FUNCTION "FC_GRP_71" : VOID
TITLE =GROUP =71
{ S7_language := '9(1) Angielski (Stany Zjednoczone)  11.01.2022  09:45:15' }
VERSION : 0.1


VAR_TEMP
  CL : "UDT_CABINET";	//CABINET LOCAL
  CR : "UDT_CABINET";	//CABINET REMOTE
  RelError : BOOL ;	//ERROR RELEASE
  RelErrorCL : BOOL ;	//ERROR RELEASE FROM CABINET LOCAL
  RelErrorCR : BOOL ;	//ERROR RELEASE FROM CABINET REMOTE
  RelControl : BOOL ;	//CONTROL RELEASE
  RelControlCL : BOOL ;	//CONTROL RELEASE FROM CABINET LOCAL
  RelControlCR : BOOL ;	//CONTROL RELEASE FROM CABINET REMOTE
  ErrorConfirm : BOOL ;	//ERROR CONFIRM
  AutoOn : BOOL ;	//AUTOMATIC ON
  AutoOff : BOOL ;	//AUTOMATIC OFF
  RelAuto : BOOL ;	//AUTOMATIC RELEASE
  TempFlapPos : WORD ;
  TempSetpoint : REAL ;
  LAMP_ON : BOOL ;
  Dummy_bin : BOOL ;
  H_REMAIN : INT ;
  M_REMAIN : INT ;
  S_REMAIN : INT ;
  PosClose : BOOL ;
END_VAR
BEGIN
NETWORK
TITLE =GLOBAL SIGNALS
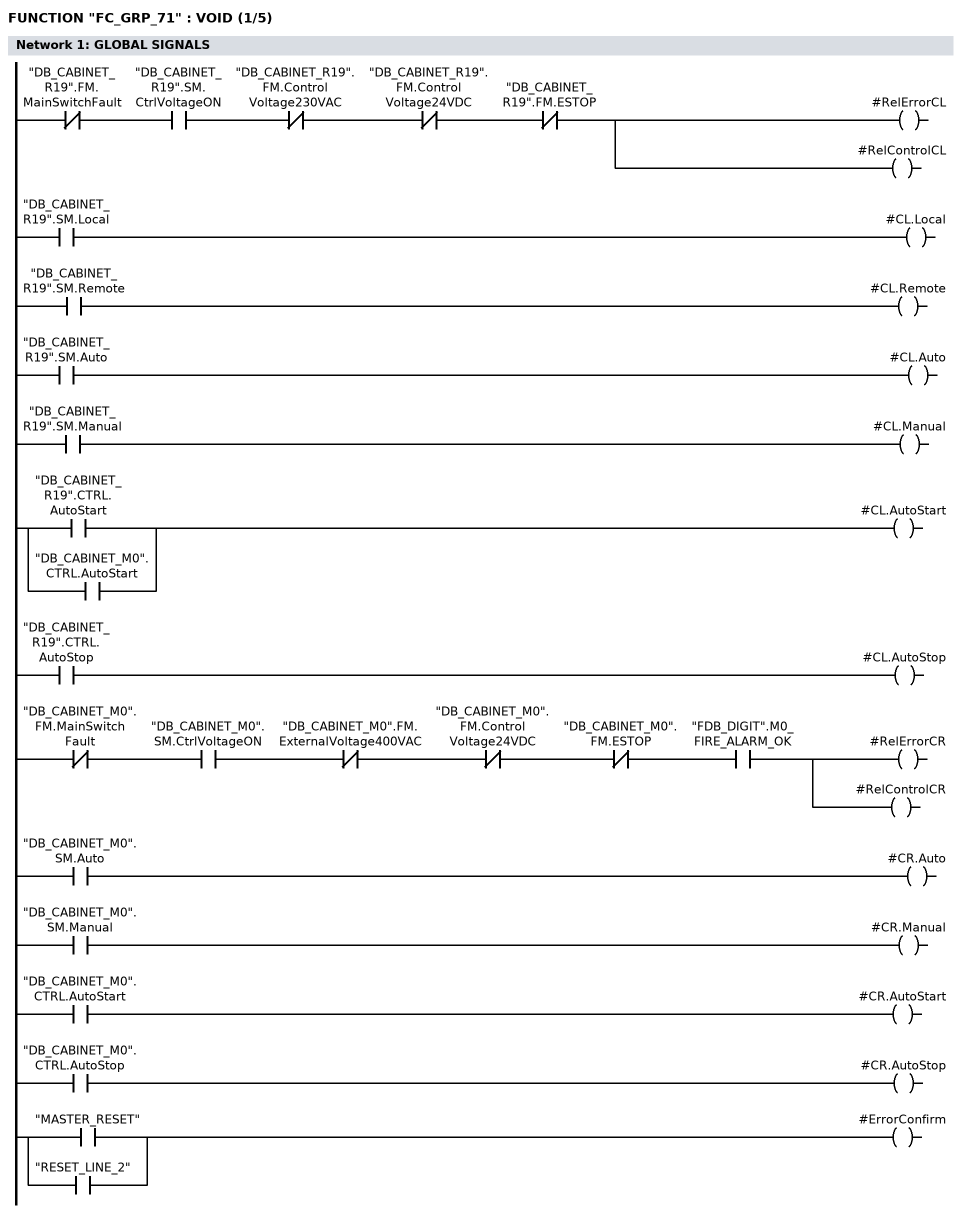
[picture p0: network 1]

//LOCAL
      UN    "DB_CABINET_R19".FM.MainSwitchFault;
      U     "DB_CABINET_R19".SM.CtrlVoltageON;
      UN    "DB_CABINET_R19".FM.ControlVoltage230VAC;
      UN    "DB_CABINET_R19".FM.ControlVoltage24VDC;
      UN    "DB_CABINET_R19".FM.ESTOP;
      =     #RelErrorCL;
      =     #RelControlCL;

      U     "DB_CABINET_R19".SM.Local;
      =     #CL.Local;
      U     "DB_CABINET_R19".SM.Remote;
      =     #CL.Remote;
      U     "DB_CABINET_R19".SM.Auto;
      =     #CL.Auto;
      U     "DB_CABINET_R19".SM.Manual;
      =     #CL.Manual;
      U     "DB_CABINET_R19".CTRL.AutoStart;
      O     "DB_CABINET_M0".CTRL.AutoStart;
      =     #CL.AutoStart;
      U     "DB_CABINET_R19".CTRL.AutoStop;
      =     #CL.AutoStop;


//REMOTE
      UN    "DB_CABINET_M0".FM.MainSwitchFault;
      U     "DB_CABINET_M0".SM.CtrlVoltageON;
      UN    "DB_CABINET_M0".FM.ExternalVoltage400VAC;
      UN    "DB_CABINET_M0".FM.ControlVoltage24VDC;
//      UN    "DB_CABINET_M0".FM.ControlVoltage230VAC_MS
      UN    "DB_CABINET_M0".FM.ESTOP;
      U     "FDB_DIGIT".M0_FIRE_ALARM_OK;
      =     #RelErrorCR;
      =     #RelControlCR;

      U     "DB_CABINET_M0".SM.Auto;
      =     #CR.Auto;
      U     "DB_CABINET_M0".SM.Manual;
      =     #CR.Manual;
      U     "DB_CABINET_M0".CTRL.AutoStart;
      =     #CR.AutoStart;
      U     "DB_CABINET_M0".CTRL.AutoStop;
      =     #CR.AutoStop;

      U     "MASTER_RESET";
      O     "RESET_LINE_2";
      =     #ErrorConfirm;

NETWORK
TITLE =GENERAL ERROR AND WARNING
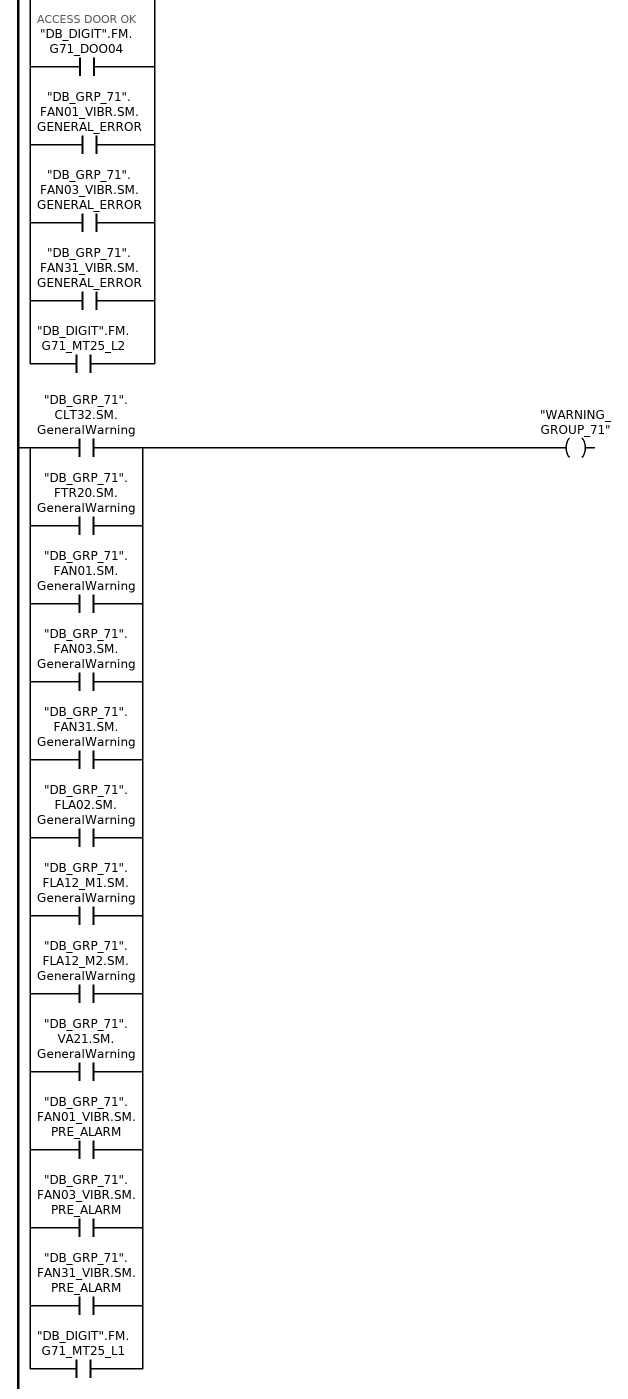
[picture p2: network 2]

      U     "DB_GRP_71".CLT32.SM.GeneralError;
      O     "DB_GRP_71".FTR20.SM.GeneralError;
      O     "DB_GRP_71".FAN01.SM.GeneralError;
      O     "DB_GRP_71".FAN03.SM.GeneralError;
      O     "DB_GRP_71".FAN31.SM.GeneralError;
      O     "DB_GRP_71".FLA02.SM.GeneralError;
      O     "DB_GRP_71".FLA12_M1.SM.GeneralError;
      O     "DB_GRP_71".FLA12_M2.SM.GeneralError;
      O     "DB_GRP_71".VA21.SM.GeneralError;
      O     "DB_DIGIT".FM.G71_FAN01; //ALARM SENSOR PRESSURE
      O     "DB_DIGIT".FM.G71_FAN03; //ALARM SENSOR PRESSURE
      O     "DB_DIGIT".FM.G71_FAN31; //ALARM SENSOR PRESSURE
      O     "DB_DIGIT".FM.G71_DOO01_FUSE; //FUSE ALARM
      O     "DB_DIGIT".FM.G71_DOO02_FUSE; //FUSE ALARM
      O     "DB_DIGIT".FM.G71_DOO03_FUSE; //FUSE ALARM
      O     "DB_DIGIT".FM.G71_DOO04_FUSE; //FUSE ALARM
      O     "DB_DIGIT".FM.G71_DOO04; // ACCESS DOOR OK
      O     "DB_GRP_71".FAN01_VIBR.SM.GENERAL_ERROR;
      O     "DB_GRP_71".FAN03_VIBR.SM.GENERAL_ERROR;
      O     "DB_GRP_71".FAN31_VIBR.SM.GENERAL_ERROR;
      O     "DB_DIGIT".FM.G71_MT25_L2;
      =     "GENERAL_FAULT_GROUP_71";


      U     "DB_GRP_71".CLT32.SM.GeneralWarning;
      O     "DB_GRP_71".FTR20.SM.GeneralWarning;
      O     "DB_GRP_71".FAN01.SM.GeneralWarning;
      O     "DB_GRP_71".FAN03.SM.GeneralWarning;
      O     "DB_GRP_71".FAN31.SM.GeneralWarning;
      O     "DB_GRP_71".FLA02.SM.GeneralWarning;
      O     "DB_GRP_71".FLA12_M1.SM.GeneralWarning;
      O     "DB_GRP_71".FLA12_M2.SM.GeneralWarning;
      O     "DB_GRP_71".VA21.SM.GeneralWarning;
      O     "DB_GRP_71".FAN01_VIBR.SM.PRE_ALARM;
      O     "DB_GRP_71".FAN03_VIBR.SM.PRE_ALARM;
      O     "DB_GRP_71".FAN31_VIBR.SM.PRE_ALARM;
      O     "DB_DIGIT".FM.G71_MT25_L1;
      =     "WARNING_GROUP_71";


NETWORK
TITLE =CONTROL/ERROR RELEASE
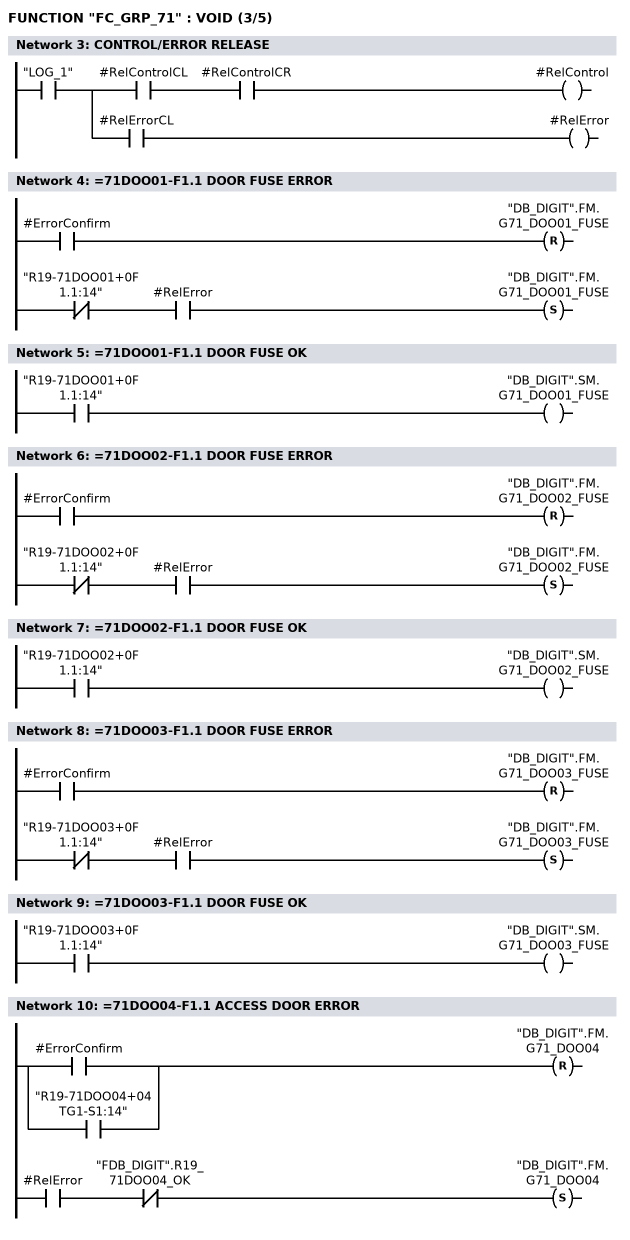
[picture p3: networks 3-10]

      U     "LOG_1";
      =     L     21.0;
      U     L     21.0;
      U     #RelControlCL;
      U     #RelControlCR;
      =     #RelControl;
      U     L     21.0;
      U     #RelErrorCL;
      =     #RelError;
NETWORK
TITLE ==71DOO01-F1.1 DOOR FUSE ERROR

      U     #ErrorConfirm;
      R     "DB_DIGIT".FM.G71_DOO01_FUSE;
      UN    "R19-71DOO01+0F1.1:14";
      U     #RelError;
      S     "DB_DIGIT".FM.G71_DOO01_FUSE;
      NOP   0;
NETWORK
TITLE ==71DOO01-F1.1 DOOR FUSE OK

      U     "R19-71DOO01+0F1.1:14";
      =     "DB_DIGIT".SM.G71_DOO01_FUSE;
NETWORK
TITLE ==71DOO02-F1.1 DOOR FUSE ERROR

      U     #ErrorConfirm;
      R     "DB_DIGIT".FM.G71_DOO02_FUSE;
      UN    "R19-71DOO02+0F1.1:14";
      U     #RelError;
      S     "DB_DIGIT".FM.G71_DOO02_FUSE;
      NOP   0;
NETWORK
TITLE ==71DOO02-F1.1 DOOR FUSE OK

      U     "R19-71DOO02+0F1.1:14";
      =     "DB_DIGIT".SM.G71_DOO02_FUSE;
NETWORK
TITLE ==71DOO03-F1.1 DOOR FUSE ERROR

      U     #ErrorConfirm;
      R     "DB_DIGIT".FM.G71_DOO03_FUSE;
      UN    "R19-71DOO03+0F1.1:14";
      U     #RelError;
      S     "DB_DIGIT".FM.G71_DOO03_FUSE;
      NOP   0;
NETWORK
TITLE ==71DOO03-F1.1 DOOR FUSE OK

      U     "R19-71DOO03+0F1.1:14";
      =     "DB_DIGIT".SM.G71_DOO03_FUSE;
NETWORK
TITLE ==71DOO04-F1.1 ACCESS DOOR ERROR

      U(    ;
      O     #ErrorConfirm;
      O     "R19-71DOO04+04TG1-S1:14";
      )     ;
      R     "DB_DIGIT".FM.G71_DOO04;
      U     #RelError;
      UN    "FDB_DIGIT".R19_71DOO04_OK;
      S     "DB_DIGIT".FM.G71_DOO04;
      NOP   0;
NETWORK
TITLE =DOOR ACKNOWLEDGEMENT
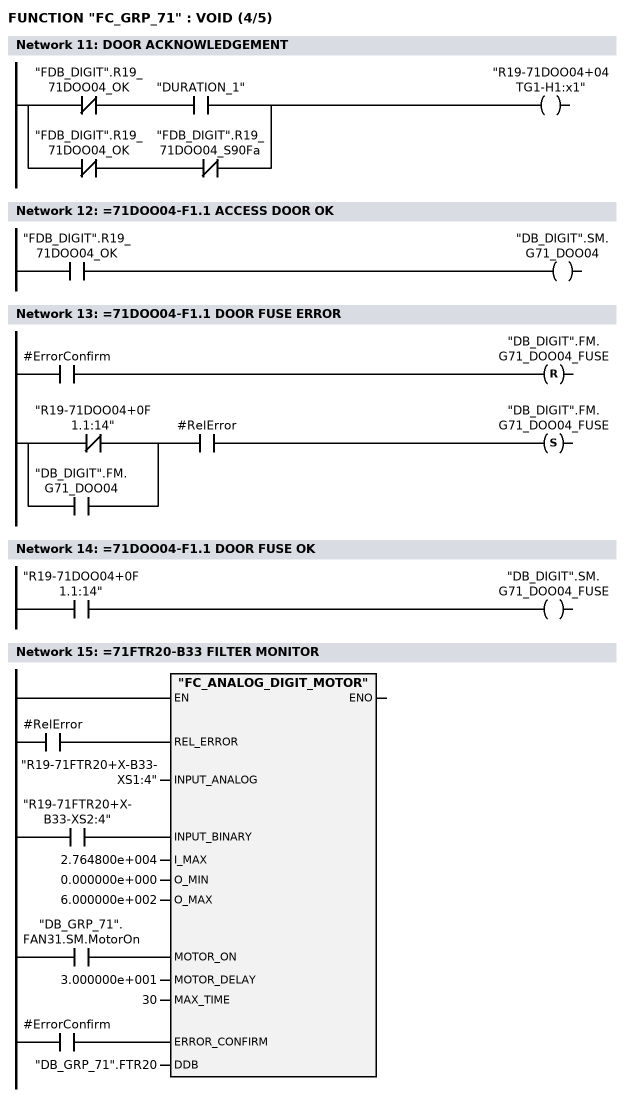
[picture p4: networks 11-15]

      UN    "FDB_DIGIT".R19_71DOO04_OK;
      U     "DURATION_1";
      O     ;
      UN    "FDB_DIGIT".R19_71DOO04_OK;
      UN    "FDB_DIGIT".R19_71DOO04_S90Fa;
      =     "R19-71DOO04+04TG1-H1:x1";
NETWORK
TITLE ==71DOO04-F1.1 ACCESS DOOR OK

      U     "FDB_DIGIT".R19_71DOO04_OK;
      =     "DB_DIGIT".SM.G71_DOO04;
NETWORK
TITLE ==71DOO04-F1.1 DOOR FUSE ERROR

      U     #ErrorConfirm;
      R     "DB_DIGIT".FM.G71_DOO04_FUSE;
      U(    ;
      ON    "R19-71DOO04+0F1.1:14";
      O     "DB_DIGIT".FM.G71_DOO04;
      )     ;
      U     #RelError;
      S     "DB_DIGIT".FM.G71_DOO04_FUSE;
      NOP   0;
NETWORK
TITLE ==71DOO04-F1.1 DOOR FUSE OK

      U     "R19-71DOO04+0F1.1:14";
      =     "DB_DIGIT".SM.G71_DOO04_FUSE;
NETWORK
TITLE ==71FTR20-B33 FILTER MONITOR

      U     #RelError;
      =     L     21.0;
      BLD   103;
      U     "R19-71FTR20+X-B33-XS2:4";
      =     L     21.1;
      BLD   103;
      U     "DB_GRP_71".FAN31.SM.MotorOn;
      =     L     21.2;
      BLD   103;
      U     #ErrorConfirm;
      =     L     21.3;
      BLD   103;
      CALL "FC_ANALOG_DIGIT_MOTOR" (
           REL_ERROR                := L     21.0,
           INPUT_ANALOG             := "R19-71FTR20+X-B33-XS1:4",
           INPUT_BINARY             := L     21.1,
           I_MAX                    := 2.764800e+004,
           O_MIN                    := 0.000000e+000,
           O_MAX                    := 6.000000e+002,
           MOTOR_ON                 := L     21.2,
           MOTOR_DELAY              := 3.000000e+001,
           MAX_TIME                 := 30,
           ERROR_CONFIRM            := L     21.3,
           DDB                      := "DB_GRP_71".FTR20);
      NOP   0;
NETWORK
TITLE ==71CLT32-B40N TEMPERATURE EXCEEDED
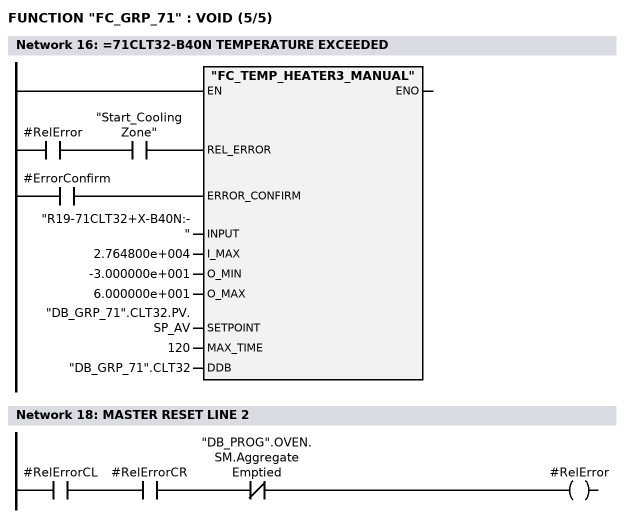
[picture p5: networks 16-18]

      U     #RelError;
      U     "Start_CoolingZone";
      =     L     21.0;
      BLD   103;
      U     #ErrorConfirm;
      =     L     21.1;
      BLD   103;
      CALL "FC_TEMP_HEATER3_MANUAL" (
           REL_ERROR                := L     21.0,
           ERROR_CONFIRM            := L     21.1,
           INPUT                    := "R19-71CLT32+X-B40N:-",
           I_MAX                    := 2.764800e+004,
           O_MIN                    := -3.000000e+001,
           O_MAX                    := 6.000000e+001,
           SETPOINT                 := "DB_GRP_71".CLT32.PV.SP_AV,
           MAX_TIME                 := 120,
           DDB                      := "DB_GRP_71".CLT32);
      NOP   0;
NETWORK
TITLE =************** FROST PROTECTION **************

NETWORK
TITLE =MASTER RESET LINE 2

      U     #RelErrorCL;
      U     #RelErrorCR;
      UN    "DB_PROG".OVEN.SM.AggregateEmptied;
      =     #RelError;
NETWORK
TITLE =FROST PROTECTION THERMOSTAT LEVEL 1, =71MT25 FAULT

      U(    ;
      O     #ErrorConfirm;
      O(    ;
      U     "R19-71MT25+K84.1:14";
      L     S5T#10S;
      SE    "T_ARES_LEV1_L2";
      NOP   0;
      NOP   0;
      NOP   0;
      U     "T_ARES_LEV1_L2";
      )     ;
      )     ;
      R     "DB_DIGIT".FM.G71_MT25_L1;
      UN    "R19-71MT25+K84.1:14";
      U     #RelError;
      S     "DB_DIGIT".FM.G71_MT25_L1;
      NOP   0;
NETWORK
TITLE =FROST PROTECTION THERMOSTAT LEVEL 1, =71MT25 FAULT
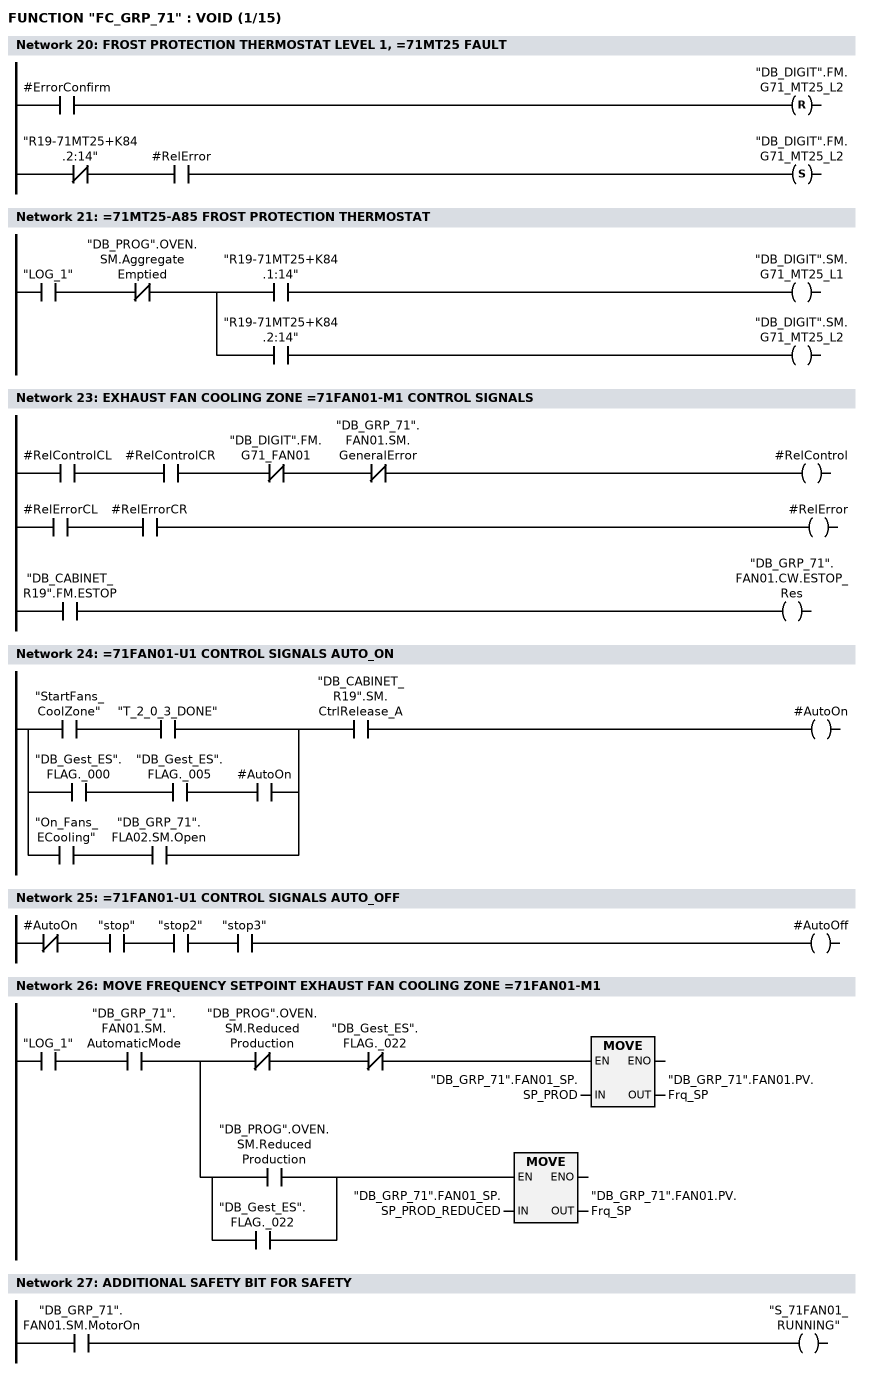
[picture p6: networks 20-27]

      U     #ErrorConfirm;
      R     "DB_DIGIT".FM.G71_MT25_L2;
      UN    "R19-71MT25+K84.2:14";
      U     #RelError;
      S     "DB_DIGIT".FM.G71_MT25_L2;
      NOP   0;
NETWORK
TITLE ==71MT25-A85 FROST PROTECTION THERMOSTAT

      U     "LOG_1";
      UN    "DB_PROG".OVEN.SM.AggregateEmptied;
      =     L     21.0;
      U     L     21.0;
      U     "R19-71MT25+K84.1:14";
      =     "DB_DIGIT".SM.G71_MT25_L1;
      U     L     21.0;
      U     "R19-71MT25+K84.2:14";
      =     "DB_DIGIT".SM.G71_MT25_L2;
NETWORK
TITLE =********* 71FAN01 ****************

NETWORK
TITLE =EXHAUST FAN COOLING ZONE =71FAN01-M1 CONTROL SIGNALS

      U     #RelControlCL;
      U     #RelControlCR;
      UN    "DB_DIGIT".FM.G71_FAN01;
      UN    "DB_GRP_71".FAN01.SM.GeneralError;
      =     #RelControl;

      U     #RelErrorCL;
      U     #RelErrorCR;
      =     #RelError;

      U     "DB_CABINET_R19".FM.ESTOP;
      =     "DB_GRP_71".FAN01.CW.ESTOP_Res;
NETWORK
TITLE ==71FAN01-U1 CONTROL SIGNALS AUTO_ON

      U(    ;
      U     "StartFans_CoolZone";
      U     "T_2_0_3_DONE";
      O     ;
      U     "DB_Gest_ES".FLAG._000;
      U     "DB_Gest_ES".FLAG._005;
      U     #AutoOn;
      O     ;
      U     "On_Fans_ECooling";
      U     "DB_GRP_71".FLA02.SM.Open;
      )     ;
      U     "DB_CABINET_R19".SM.CtrlRelease_A;
      =     #AutoOn;
NETWORK
TITLE ==71FAN01-U1 CONTROL SIGNALS AUTO_OFF

      UN    #AutoOn;
      U     "stop";
      U     "stop2";
      U     "stop3";
      =     #AutoOff;
NETWORK
TITLE =MOVE FREQUENCY SETPOINT EXHAUST FAN COOLING ZONE =71FAN01-M1

      U     "LOG_1";
      U     "DB_GRP_71".FAN01.SM.AutomaticMode;
      =     L     21.0;
      U     L     21.0;
      UN    "DB_PROG".OVEN.SM.ReducedProduction;
      UN    "DB_Gest_ES".FLAG._022;
      SPBNB _001;
      L     "DB_GRP_71".FAN01_SP.SP_PROD;
      T     "DB_GRP_71".FAN01.PV.Frq_SP;
_001: NOP   0;
      U     L     21.0;
      U(    ;
      O     "DB_PROG".OVEN.SM.ReducedProduction;
      O     "DB_Gest_ES".FLAG._022;
      )     ;
      SPBNB _002;
      L     "DB_GRP_71".FAN01_SP.SP_PROD_REDUCED;
      T     "DB_GRP_71".FAN01.PV.Frq_SP;
_002: NOP   0;
NETWORK
TITLE =ADDITIONAL SAFETY BIT FOR SAFETY

      U     "DB_GRP_71".FAN01.SM.MotorOn;
      =     "S_71FAN01_RUNNING";
NETWORK
TITLE =ON/START
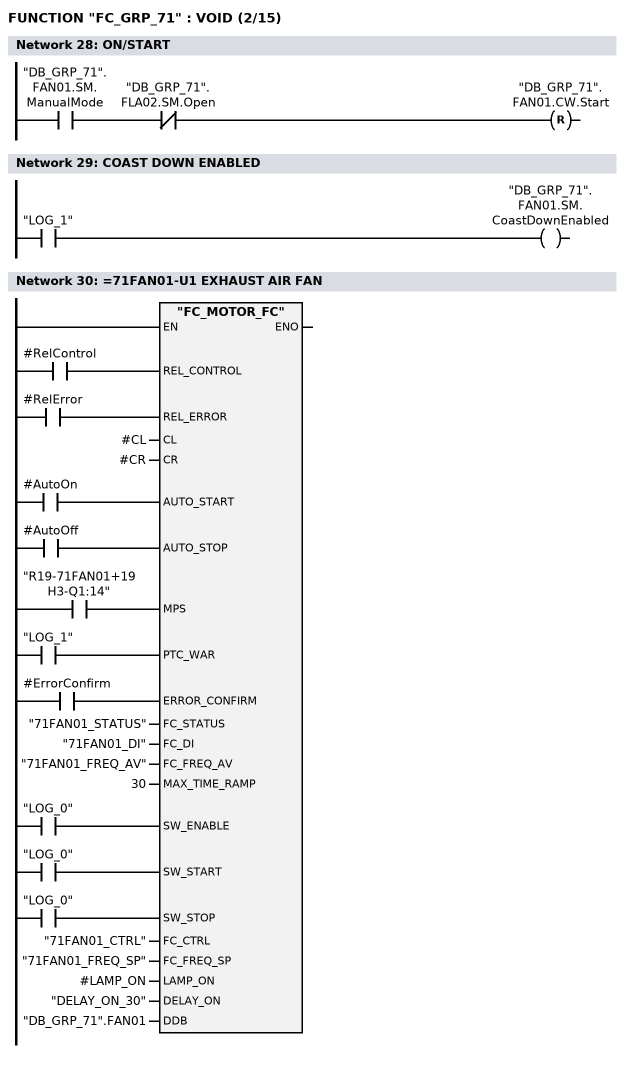
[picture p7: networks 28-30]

      U     "DB_GRP_71".FAN01.SM.ManualMode;
      UN    "DB_GRP_71".FLA02.SM.Open;
      R     "DB_GRP_71".FAN01.CW.Start;
NETWORK
TITLE =COAST DOWN ENABLED

      U     "LOG_1";
      =     "DB_GRP_71".FAN01.SM.CoastDownEnabled;
NETWORK
TITLE ==71FAN01-U1 EXHAUST AIR FAN

      U     #RelControl;
      =     L     21.0;
      BLD   103;
      U     #RelError;
      =     L     21.1;
      BLD   103;
      U     #AutoOn;
      =     L     21.2;
      BLD   103;
      U     #AutoOff;
      =     L     21.3;
      BLD   103;
      U     "R19-71FAN01+19H3-Q1:14";
      =     L     21.4;
      BLD   103;
      U     "LOG_1";
      =     L     21.5;
      BLD   103;
      U     #ErrorConfirm;
      =     L     21.6;
      BLD   103;
      U     "LOG_0";
      =     L     21.7;
      BLD   103;
      U     "LOG_0";
      =     L     22.0;
      BLD   103;
      U     "LOG_0";
      =     L     22.1;
      BLD   103;
      CALL "FC_MOTOR_FC" (
           REL_CONTROL              := L     21.0,
           REL_ERROR                := L     21.1,
           CL                       := #CL,
           CR                       := #CR,
           AUTO_START               := L     21.2,
           AUTO_STOP                := L     21.3,
           MPS                      := L     21.4,
           PTC_WAR                  := L     21.5,
           ERROR_CONFIRM            := L     21.6,
           FC_STATUS                := "71FAN01_STATUS",
           FC_DI                    := "71FAN01_DI",
           FC_FREQ_AV               := "71FAN01_FREQ_AV",
           MAX_TIME_RAMP            := 30,
           SW_ENABLE                := L     21.7,
           SW_START                 := L     22.0,
           SW_STOP                  := L     22.1,
           FC_CTRL                  := "71FAN01_CTRL",
           FC_FREQ_SP               := "71FAN01_FREQ_SP",
           LAMP_ON                  := #LAMP_ON,
           DELAY_ON                 := "DELAY_ON_30",
           DDB                      := "DB_GRP_71".FAN01);
      NOP   0;
NETWORK
TITLE ==71FAN01-S32F  CONTROL PRESSURE
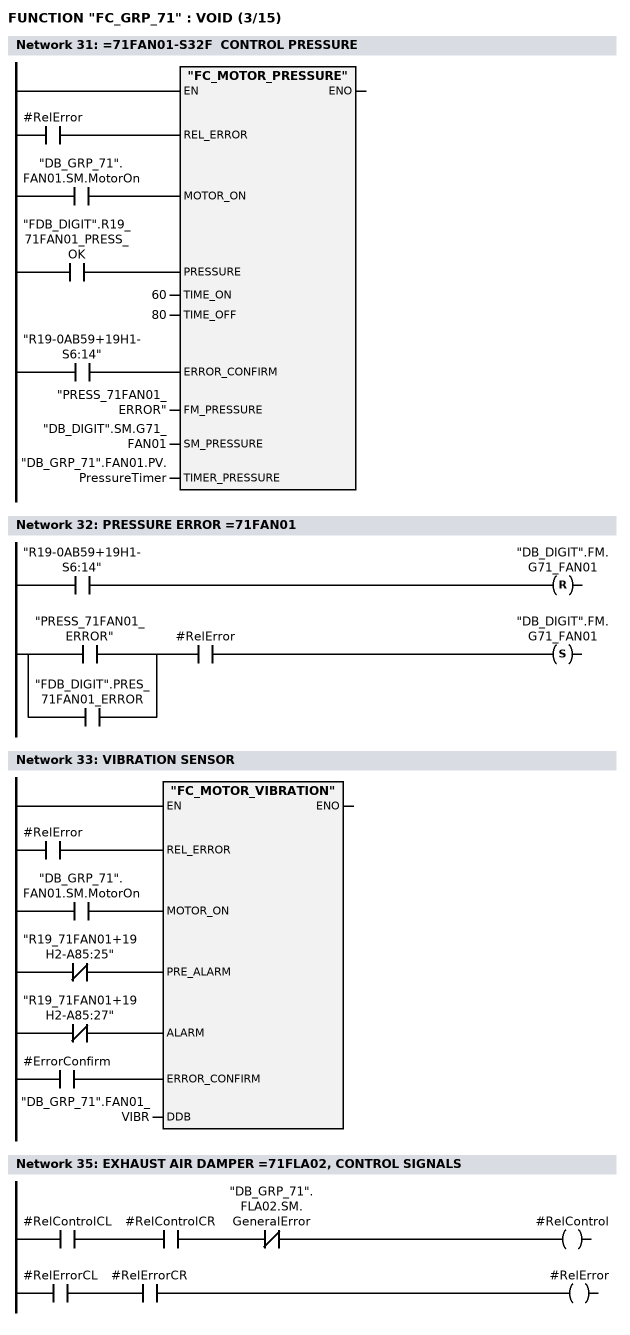
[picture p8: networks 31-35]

      U     #RelError;
      =     L     21.0;
      BLD   103;
      U     "DB_GRP_71".FAN01.SM.MotorOn;
      =     L     21.1;
      BLD   103;
      U     "FDB_DIGIT".R19_71FAN01_PRESS_OK;
      =     L     21.2;
      BLD   103;
      U     "R19-0AB59+19H1-S6:14";
      =     L     21.3;
      BLD   103;
      CALL "FC_MOTOR_PRESSURE" (
           REL_ERROR                := L     21.0,
           MOTOR_ON                 := L     21.1,
           PRESSURE                 := L     21.2,
           TIME_ON                  := 60,
           TIME_OFF                 := 80,
           ERROR_CONFIRM            := L     21.3,
           FM_PRESSURE              := "PRESS_71FAN01_ERROR",
           SM_PRESSURE              := "DB_DIGIT".SM.G71_FAN01,
           TIMER_PRESSURE           := "DB_GRP_71".FAN01.PV.PressureTimer);
      NOP   0;
NETWORK
TITLE =PRESSURE ERROR =71FAN01

      U     "R19-0AB59+19H1-S6:14";
      R     "DB_DIGIT".FM.G71_FAN01;
      U(    ;
      O     "PRESS_71FAN01_ERROR";
      O     "FDB_DIGIT".PRES_71FAN01_ERROR;
      )     ;
      U     #RelError;
      S     "DB_DIGIT".FM.G71_FAN01;
      NOP   0;
NETWORK
TITLE =VIBRATION SENSOR

      U     #RelError;
      =     L     21.0;
      BLD   103;
      U     "DB_GRP_71".FAN01.SM.MotorOn;
      =     L     21.1;
      BLD   103;
      UN    "R19_71FAN01+19H2-A85:25";
      =     L     21.2;
      BLD   103;
      UN    "R19_71FAN01+19H2-A85:27";
      =     L     21.3;
      BLD   103;
      U     #ErrorConfirm;
      =     L     21.4;
      BLD   103;
      CALL "FC_MOTOR_VIBRATION" (
           REL_ERROR                := L     21.0,
           MOTOR_ON                 := L     21.1,
           PRE_ALARM                := L     21.2,
           ALARM                    := L     21.3,
           ERROR_CONFIRM            := L     21.4,
           DDB                      := "DB_GRP_71".FAN01_VIBR);
      NOP   0;
NETWORK
TITLE =*********** 71FLA02 ***********

NETWORK
TITLE =EXHAUST AIR DAMPER =71FLA02, CONTROL SIGNALS

      U     #RelControlCL;
      U     #RelControlCR;
      UN    "DB_GRP_71".FLA02.SM.GeneralError;
      =     #RelControl;



      U     #RelErrorCL;
      U     #RelErrorCR;
      =     #RelError;



NETWORK
TITLE =PAUSE CLOSE FLAP =71FLA02
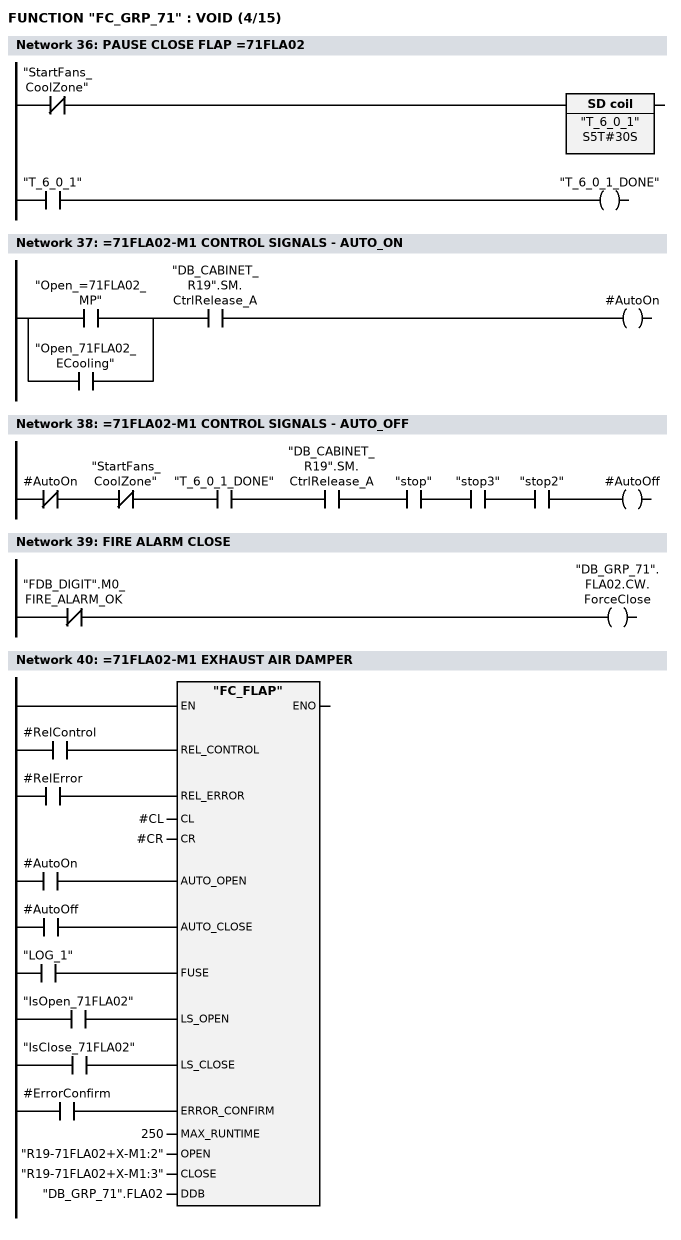
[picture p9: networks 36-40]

      UN    "StartFans_CoolZone";
      L     S5T#30S;
      SE    "T_6_0_1";
      NOP   0;
      NOP   0;
      NOP   0;
      U     "T_6_0_1";
      =     "T_6_0_1_DONE";
NETWORK
TITLE ==71FLA02-M1 CONTROL SIGNALS - AUTO_ON

      U(    ;
      O     "Open_=71FLA02_MP";
      O     "Open_71FLA02_ECooling";
      )     ;
      U     "DB_CABINET_R19".SM.CtrlRelease_A;
      =     #AutoOn;
NETWORK
TITLE ==71FLA02-M1 CONTROL SIGNALS - AUTO_OFF

      UN    #AutoOn;
      UN    "StartFans_CoolZone";
      U     "T_6_0_1_DONE";
      U     "DB_CABINET_R19".SM.CtrlRelease_A;
      U     "stop";
      U     "stop3";
      U     "stop2";
      =     #AutoOff;
NETWORK
TITLE =FIRE ALARM CLOSE

      UN    "FDB_DIGIT".M0_FIRE_ALARM_OK;
      =     "DB_GRP_71".FLA02.CW.ForceClose;
NETWORK
TITLE ==71FLA02-M1 EXHAUST AIR DAMPER

      U     #RelControl;
      =     L     21.0;
      BLD   103;
      U     #RelError;
      =     L     21.1;
      BLD   103;
      U     #AutoOn;
      =     L     21.2;
      BLD   103;
      U     #AutoOff;
      =     L     21.3;
      BLD   103;
      U     "LOG_1";
      =     L     21.4;
      BLD   103;
      U     "IsOpen_71FLA02";
      =     L     21.5;
      BLD   103;
      U     "IsClose_71FLA02";
      =     L     21.6;
      BLD   103;
      U     #ErrorConfirm;
      =     L     21.7;
      BLD   103;
      CALL "FC_FLAP" (
           REL_CONTROL              := L     21.0,
           REL_ERROR                := L     21.1,
           CL                       := #CL,
           CR                       := #CR,
           AUTO_OPEN                := L     21.2,
           AUTO_CLOSE               := L     21.3,
           FUSE                     := L     21.4,
           LS_OPEN                  := L     21.5,
           LS_CLOSE                 := L     21.6,
           ERROR_CONFIRM            := L     21.7,
           MAX_RUNTIME              := 250,
           OPEN                     := "R19-71FLA02+X-M1:2",
           CLOSE                    := "R19-71FLA02+X-M1:3",
           DDB                      := "DB_GRP_71".FLA02);
      NOP   0;
NETWORK
TITLE ==71FLA02-M1 EXHAUST AIR DAMPER POSITION
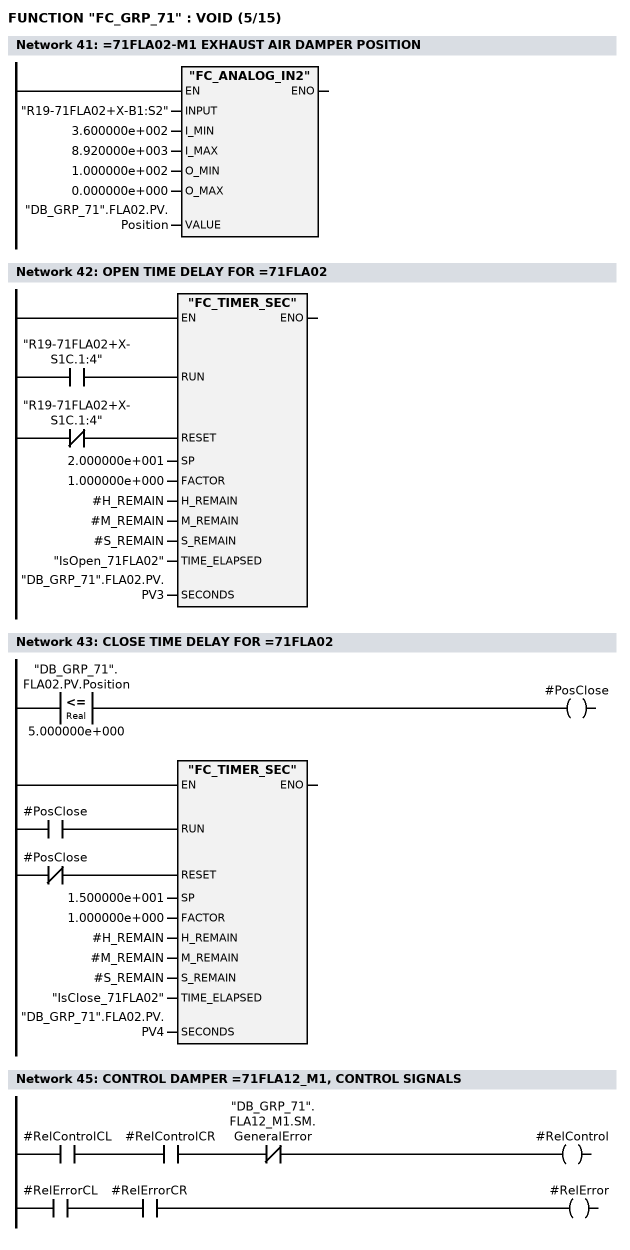
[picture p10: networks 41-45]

      CALL "FC_ANALOG_IN2" (
           INPUT                    := "R19-71FLA02+X-B1:S2",
           I_MIN                    := 3.600000e+002,
           I_MAX                    := 8.920000e+003,
           O_MIN                    := 1.000000e+002,
           O_MAX                    := 0.000000e+000,
           VALUE                    := "DB_GRP_71".FLA02.PV.Position);
      NOP   0;
NETWORK
TITLE =OPEN TIME DELAY FOR =71FLA02

      U     "R19-71FLA02+X-S1C.1:4";
      =     L     21.0;
      BLD   103;
      UN    "R19-71FLA02+X-S1C.1:4";
      =     L     21.1;
      BLD   103;
      CALL "FC_TIMER_SEC" (
           RUN                      := L     21.0,
           RESET                    := L     21.1,
           SP                       := 2.000000e+001,
           FACTOR                   := 1.000000e+000,
           H_REMAIN                 := #H_REMAIN,
           M_REMAIN                 := #M_REMAIN,
           S_REMAIN                 := #S_REMAIN,
           TIME_ELAPSED             := "IsOpen_71FLA02",
           SECONDS                  := "DB_GRP_71".FLA02.PV.PV3);
      NOP   0;
NETWORK
TITLE =CLOSE TIME DELAY FOR =71FLA02

      U(    ;
      L     "DB_GRP_71".FLA02.PV.Position;
      L     5.000000e+000;
      <=R   ;
      )     ;
      =     #PosClose;
      U     #PosClose;
      =     L     21.0;
      BLD   103;
      UN    #PosClose;
      =     L     21.1;
      BLD   103;
      CALL "FC_TIMER_SEC" (
           RUN                      := L     21.0,
           RESET                    := L     21.1,
           SP                       := 1.500000e+001,
           FACTOR                   := 1.000000e+000,
           H_REMAIN                 := #H_REMAIN,
           M_REMAIN                 := #M_REMAIN,
           S_REMAIN                 := #S_REMAIN,
           TIME_ELAPSED             := "IsClose_71FLA02",
           SECONDS                  := "DB_GRP_71".FLA02.PV.PV4);
      NOP   0;
NETWORK
TITLE =************ 71FLA12_M1 *******************

NETWORK
TITLE =CONTROL DAMPER =71FLA12_M1, CONTROL SIGNALS

      U     #RelControlCL;
      U     #RelControlCR;
      UN    "DB_GRP_71".FLA12_M1.SM.GeneralError;
      =     #RelControl;


      U     #RelErrorCL;
      U     #RelErrorCR;
      =     #RelError;


NETWORK
TITLE ==71FLA12_M1 CONTROL SIGNALS - AUTO_ON
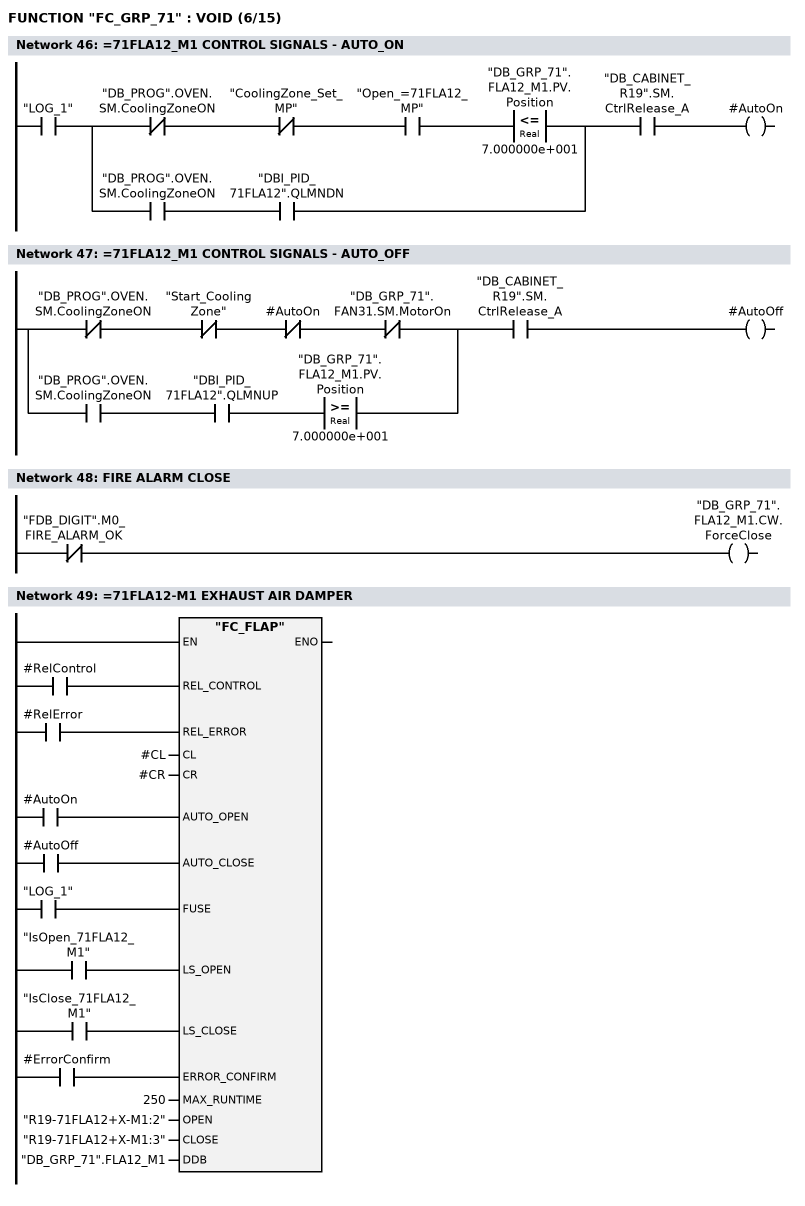
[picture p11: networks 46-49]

      U     "LOG_1";
      U(    ;
      UN    "DB_PROG".OVEN.SM.CoolingZoneON;
      UN    "CoolingZone_Set_MP";
      U     "Open_=71FLA12_MP";
      U(    ;
      L     "DB_GRP_71".FLA12_M1.PV.Position;
      L     7.000000e+001;
      <=R   ;
      )     ;
      O     ;
      U     "DB_PROG".OVEN.SM.CoolingZoneON;
      U     "DBI_PID_71FLA12".QLMNDN;
      )     ;
      U     "DB_CABINET_R19".SM.CtrlRelease_A;
      =     #AutoOn;
NETWORK
TITLE ==71FLA12_M1 CONTROL SIGNALS - AUTO_OFF

      U(    ;
      UN    "DB_PROG".OVEN.SM.CoolingZoneON;
      UN    "Start_CoolingZone";
      UN    #AutoOn;
      UN    "DB_GRP_71".FAN31.SM.MotorOn;
      O     ;
      U     "DB_PROG".OVEN.SM.CoolingZoneON;
      U     "DBI_PID_71FLA12".QLMNUP;
      U(    ;
      L     "DB_GRP_71".FLA12_M1.PV.Position;
      L     7.000000e+001;
      >=R   ;
      )     ;
      )     ;
      U     "DB_CABINET_R19".SM.CtrlRelease_A;
      =     #AutoOff;
NETWORK
TITLE =FIRE ALARM CLOSE

      UN    "FDB_DIGIT".M0_FIRE_ALARM_OK;
      =     "DB_GRP_71".FLA12_M1.CW.ForceClose;
NETWORK
TITLE ==71FLA12-M1 EXHAUST AIR DAMPER

      U     #RelControl;
      =     L     21.0;
      BLD   103;
      U     #RelError;
      =     L     21.1;
      BLD   103;
      U     #AutoOn;
      =     L     21.2;
      BLD   103;
      U     #AutoOff;
      =     L     21.3;
      BLD   103;
      U     "LOG_1";
      =     L     21.4;
      BLD   103;
      U     "IsOpen_71FLA12_M1";
      =     L     21.5;
      BLD   103;
      U     "IsClose_71FLA12_M1";
      =     L     21.6;
      BLD   103;
      U     #ErrorConfirm;
      =     L     21.7;
      BLD   103;
      CALL "FC_FLAP" (
           REL_CONTROL              := L     21.0,
           REL_ERROR                := L     21.1,
           CL                       := #CL,
           CR                       := #CR,
           AUTO_OPEN                := L     21.2,
           AUTO_CLOSE               := L     21.3,
           FUSE                     := L     21.4,
           LS_OPEN                  := L     21.5,
           LS_CLOSE                 := L     21.6,
           ERROR_CONFIRM            := L     21.7,
           MAX_RUNTIME              := 250,
           OPEN                     := "R19-71FLA12+X-M1:2",
           CLOSE                    := "R19-71FLA12+X-M1:3",
           DDB                      := "DB_GRP_71".FLA12_M1);
      NOP   0;
NETWORK
TITLE =OPEN TIME DELAY FOR =71FLA12_M1
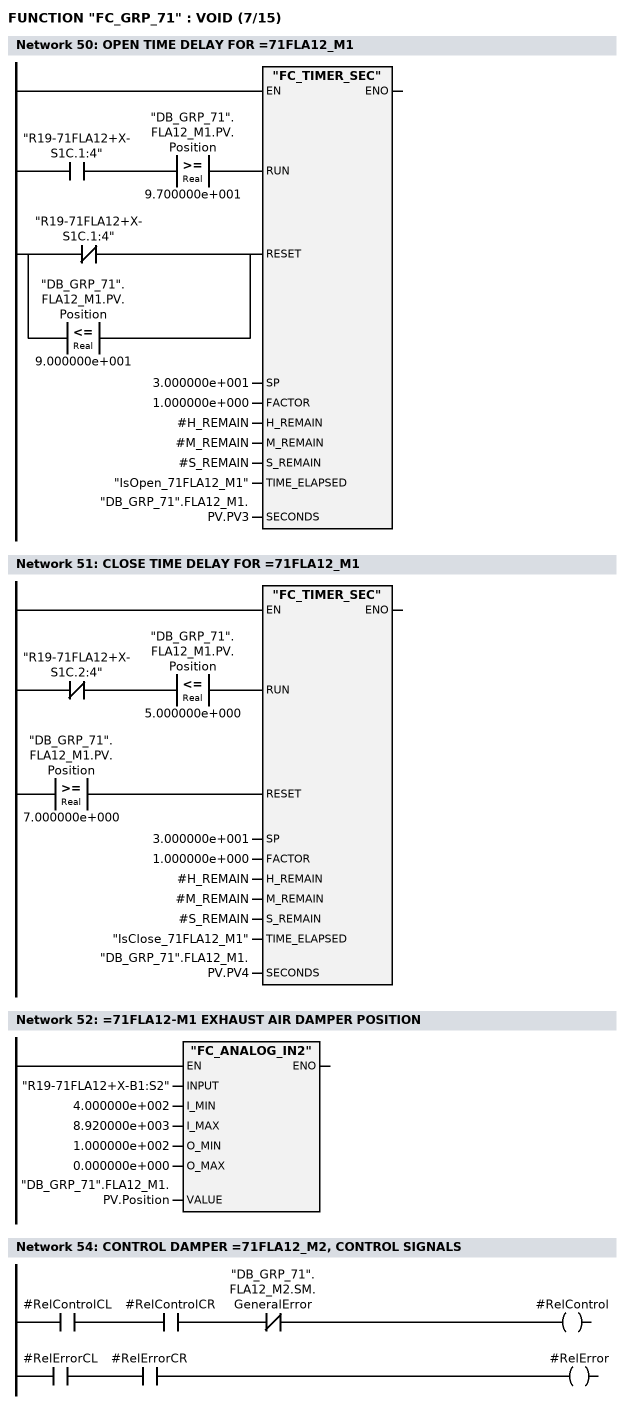
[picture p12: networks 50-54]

      U     "R19-71FLA12+X-S1C.1:4";
      U(    ;
      L     "DB_GRP_71".FLA12_M1.PV.Position;
      L     9.700000e+001;
      >=R   ;
      )     ;
      =     L     21.0;
      BLD   103;
      U(    ;
      ON    "R19-71FLA12+X-S1C.1:4";
      O(    ;
      L     "DB_GRP_71".FLA12_M1.PV.Position;
      L     9.000000e+001;
      <=R   ;
      )     ;
      )     ;
      =     L     21.1;
      BLD   103;
      CALL "FC_TIMER_SEC" (
           RUN                      := L     21.0,
           RESET                    := L     21.1,
           SP                       := 3.000000e+001,
           FACTOR                   := 1.000000e+000,
           H_REMAIN                 := #H_REMAIN,
           M_REMAIN                 := #M_REMAIN,
           S_REMAIN                 := #S_REMAIN,
           TIME_ELAPSED             := "IsOpen_71FLA12_M1",
           SECONDS                  := "DB_GRP_71".FLA12_M1.PV.PV3);
      NOP   0;
NETWORK
TITLE =CLOSE TIME DELAY FOR =71FLA12_M1

      UN    "R19-71FLA12+X-S1C.2:4";
      U(    ;
      L     "DB_GRP_71".FLA12_M1.PV.Position;
      L     5.000000e+000;
      <=R   ;
      )     ;
      =     L     21.0;
      BLD   103;
      U(    ;
      L     "DB_GRP_71".FLA12_M1.PV.Position;
      L     7.000000e+000;
      >=R   ;
      )     ;
      =     L     21.1;
      BLD   103;
      CALL "FC_TIMER_SEC" (
           RUN                      := L     21.0,
           RESET                    := L     21.1,
           SP                       := 3.000000e+001,
           FACTOR                   := 1.000000e+000,
           H_REMAIN                 := #H_REMAIN,
           M_REMAIN                 := #M_REMAIN,
           S_REMAIN                 := #S_REMAIN,
           TIME_ELAPSED             := "IsClose_71FLA12_M1",
           SECONDS                  := "DB_GRP_71".FLA12_M1.PV.PV4);
      NOP   0;
NETWORK
TITLE ==71FLA12-M1 EXHAUST AIR DAMPER POSITION

      CALL "FC_ANALOG_IN2" (
           INPUT                    := "R19-71FLA12+X-B1:S2",
           I_MIN                    := 4.000000e+002,
           I_MAX                    := 8.920000e+003,
           O_MIN                    := 1.000000e+002,
           O_MAX                    := 0.000000e+000,
           VALUE                    := "DB_GRP_71".FLA12_M1.PV.Position);
      NOP   0;
NETWORK
TITLE =**************** 71FLA12_M2 *****************

NETWORK
TITLE =CONTROL DAMPER =71FLA12_M2, CONTROL SIGNALS

      U     #RelControlCL;
      U     #RelControlCR;
      UN    "DB_GRP_71".FLA12_M2.SM.GeneralError;
      =     #RelControl;


      U     #RelErrorCL;
      U     #RelErrorCR;
      =     #RelError;


NETWORK
TITLE ==71FLA12_M2 CONTROL SIGNALS - AUTO_ON
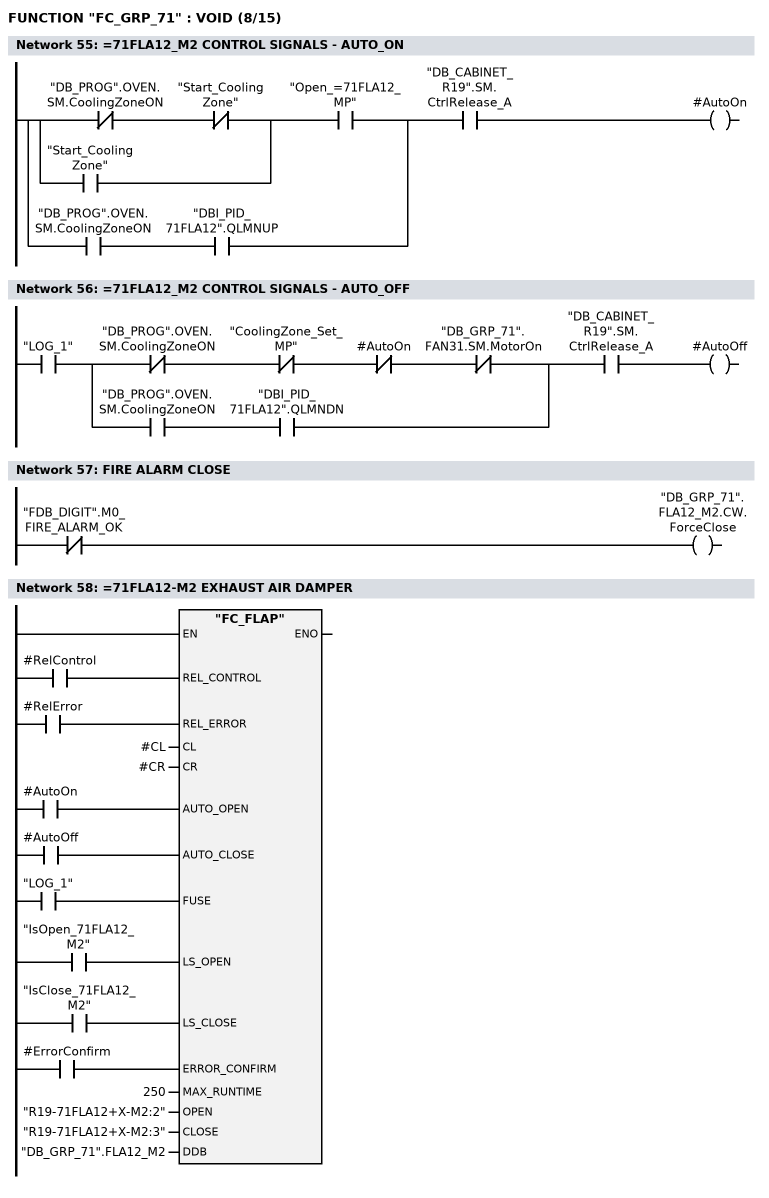
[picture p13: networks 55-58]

      U(    ;
      U(    ;
      UN    "DB_PROG".OVEN.SM.CoolingZoneON;
      UN    "Start_CoolingZone";
      O     "Start_CoolingZone";
      )     ;
      U     "Open_=71FLA12_MP";
      O     ;
      U     "DB_PROG".OVEN.SM.CoolingZoneON;
      U     "DBI_PID_71FLA12".QLMNUP;
      )     ;
      U     "DB_CABINET_R19".SM.CtrlRelease_A;
      =     #AutoOn;
NETWORK
TITLE ==71FLA12_M2 CONTROL SIGNALS - AUTO_OFF

      U     "LOG_1";
      U(    ;
      UN    "DB_PROG".OVEN.SM.CoolingZoneON;
      UN    "CoolingZone_Set_MP";
      UN    #AutoOn;
      UN    "DB_GRP_71".FAN31.SM.MotorOn;
      O     ;
      U     "DB_PROG".OVEN.SM.CoolingZoneON;
      U     "DBI_PID_71FLA12".QLMNDN;
      )     ;
      U     "DB_CABINET_R19".SM.CtrlRelease_A;
      =     #AutoOff;
NETWORK
TITLE =FIRE ALARM CLOSE

      UN    "FDB_DIGIT".M0_FIRE_ALARM_OK;
      =     "DB_GRP_71".FLA12_M2.CW.ForceClose;
NETWORK
TITLE ==71FLA12-M2 EXHAUST AIR DAMPER

      U     #RelControl;
      =     L     21.0;
      BLD   103;
      U     #RelError;
      =     L     21.1;
      BLD   103;
      U     #AutoOn;
      =     L     21.2;
      BLD   103;
      U     #AutoOff;
      =     L     21.3;
      BLD   103;
      U     "LOG_1";
      =     L     21.4;
      BLD   103;
      U     "IsOpen_71FLA12_M2";
      =     L     21.5;
      BLD   103;
      U     "IsClose_71FLA12_M2";
      =     L     21.6;
      BLD   103;
      U     #ErrorConfirm;
      =     L     21.7;
      BLD   103;
      CALL "FC_FLAP" (
           REL_CONTROL              := L     21.0,
           REL_ERROR                := L     21.1,
           CL                       := #CL,
           CR                       := #CR,
           AUTO_OPEN                := L     21.2,
           AUTO_CLOSE               := L     21.3,
           FUSE                     := L     21.4,
           LS_OPEN                  := L     21.5,
           LS_CLOSE                 := L     21.6,
           ERROR_CONFIRM            := L     21.7,
           MAX_RUNTIME              := 250,
           OPEN                     := "R19-71FLA12+X-M2:2",
           CLOSE                    := "R19-71FLA12+X-M2:3",
           DDB                      := "DB_GRP_71".FLA12_M2);
      NOP   0;
NETWORK
TITLE =OPEN TIME DELAY FOR =71FLA12_M2
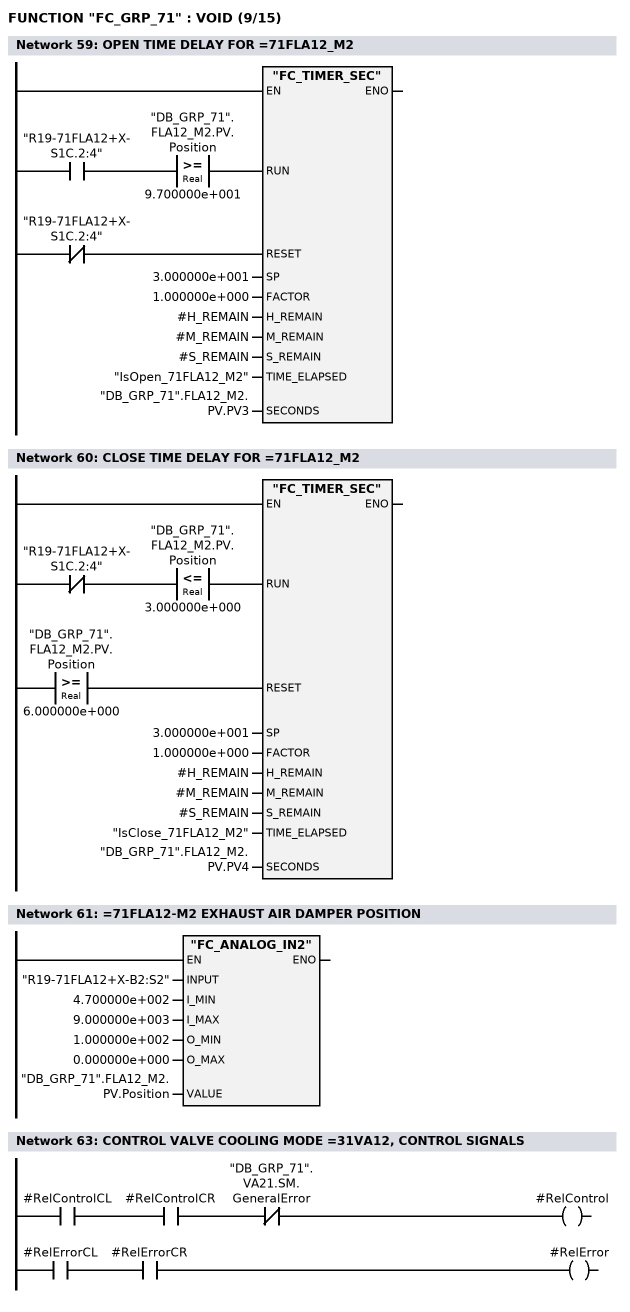
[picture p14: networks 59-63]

      U     "R19-71FLA12+X-S1C.2:4";
      U(    ;
      L     "DB_GRP_71".FLA12_M2.PV.Position;
      L     9.700000e+001;
      >=R   ;
      )     ;
      =     L     21.0;
      BLD   103;
      UN    "R19-71FLA12+X-S1C.2:4";
      =     L     21.1;
      BLD   103;
      CALL "FC_TIMER_SEC" (
           RUN                      := L     21.0,
           RESET                    := L     21.1,
           SP                       := 3.000000e+001,
           FACTOR                   := 1.000000e+000,
           H_REMAIN                 := #H_REMAIN,
           M_REMAIN                 := #M_REMAIN,
           S_REMAIN                 := #S_REMAIN,
           TIME_ELAPSED             := "IsOpen_71FLA12_M2",
           SECONDS                  := "DB_GRP_71".FLA12_M2.PV.PV3);
      NOP   0;
NETWORK
TITLE =CLOSE TIME DELAY FOR =71FLA12_M2

      UN    "R19-71FLA12+X-S1C.2:4";
      U(    ;
      L     "DB_GRP_71".FLA12_M2.PV.Position;
      L     3.000000e+000;
      <=R   ;
      )     ;
      =     L     21.0;
      BLD   103;
      U(    ;
      L     "DB_GRP_71".FLA12_M2.PV.Position;
      L     6.000000e+000;
      >=R   ;
      )     ;
      =     L     21.1;
      BLD   103;
      CALL "FC_TIMER_SEC" (
           RUN                      := L     21.0,
           RESET                    := L     21.1,
           SP                       := 3.000000e+001,
           FACTOR                   := 1.000000e+000,
           H_REMAIN                 := #H_REMAIN,
           M_REMAIN                 := #M_REMAIN,
           S_REMAIN                 := #S_REMAIN,
           TIME_ELAPSED             := "IsClose_71FLA12_M2",
           SECONDS                  := "DB_GRP_71".FLA12_M2.PV.PV4);
      NOP   0;
NETWORK
TITLE ==71FLA12-M2 EXHAUST AIR DAMPER POSITION

      CALL "FC_ANALOG_IN2" (
           INPUT                    := "R19-71FLA12+X-B2:S2",
           I_MIN                    := 4.700000e+002,
           I_MAX                    := 9.000000e+003,
           O_MIN                    := 1.000000e+002,
           O_MAX                    := 0.000000e+000,
           VALUE                    := "DB_GRP_71".FLA12_M2.PV.Position);
      NOP   0;
NETWORK
TITLE =********** 31VA12 *********************

NETWORK
TITLE =CONTROL VALVE COOLING MODE =31VA12, CONTROL SIGNALS

      U     #RelControlCL;
      U     #RelControlCR;
      UN    "DB_GRP_71".VA21.SM.GeneralError;
      =     #RelControl;

      U     #RelErrorCL;
      U     #RelErrorCR;
      =     #RelError;




NETWORK
TITLE =RELEASE =71VA21
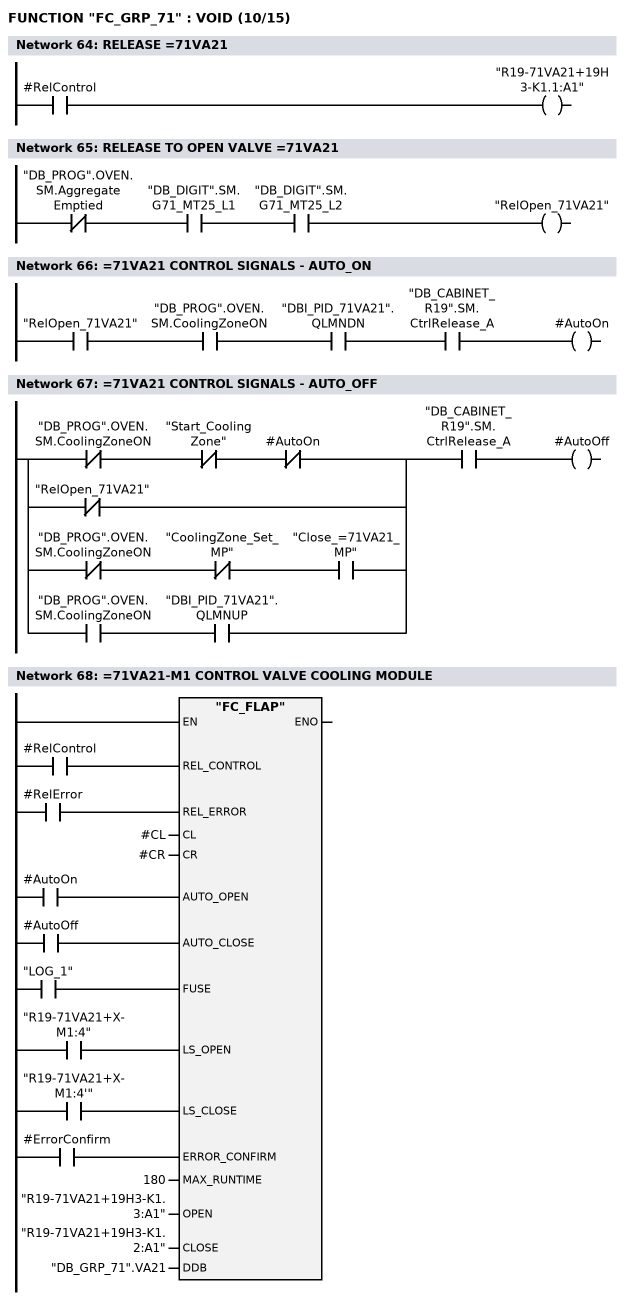
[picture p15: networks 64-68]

      U     #RelControl;
      =     "R19-71VA21+19H3-K1.1:A1";
NETWORK
TITLE =RELEASE TO OPEN VALVE =71VA21

      UN    "DB_PROG".OVEN.SM.AggregateEmptied;
      U     "DB_DIGIT".SM.G71_MT25_L1;
      U     "DB_DIGIT".SM.G71_MT25_L2;
      =     "RelOpen_71VA21";
NETWORK
TITLE ==71VA21 CONTROL SIGNALS - AUTO_ON

      U     "RelOpen_71VA21";
      U     "DB_PROG".OVEN.SM.CoolingZoneON;
      U     "DBI_PID_71VA21".QLMNDN;
      U     "DB_CABINET_R19".SM.CtrlRelease_A;
      =     #AutoOn;
NETWORK
TITLE ==71VA21 CONTROL SIGNALS - AUTO_OFF

      U(    ;
      UN    "DB_PROG".OVEN.SM.CoolingZoneON;
      UN    "Start_CoolingZone";
      UN    #AutoOn;
      ON    "RelOpen_71VA21";
      O     ;
      UN    "DB_PROG".OVEN.SM.CoolingZoneON;
      UN    "CoolingZone_Set_MP";
      U     "Close_=71VA21_MP";
      O     ;
      U     "DB_PROG".OVEN.SM.CoolingZoneON;
      U     "DBI_PID_71VA21".QLMNUP;
      )     ;
      U     "DB_CABINET_R19".SM.CtrlRelease_A;
      =     #AutoOff;
NETWORK
TITLE ==71VA21-M1 CONTROL VALVE COOLING MODULE

      U     #RelControl;
      =     L     21.0;
      BLD   103;
      U     #RelError;
      =     L     21.1;
      BLD   103;
      U     #AutoOn;
      =     L     21.2;
      BLD   103;
      U     #AutoOff;
      =     L     21.3;
      BLD   103;
      U     "LOG_1";
      =     L     21.4;
      BLD   103;
      U     "R19-71VA21+X-M1:4";
      =     L     21.5;
      BLD   103;
      U     "R19-71VA21+X-M1:4'";
      =     L     21.6;
      BLD   103;
      U     #ErrorConfirm;
      =     L     21.7;
      BLD   103;
      CALL "FC_FLAP" (
           REL_CONTROL              := L     21.0,
           REL_ERROR                := L     21.1,
           CL                       := #CL,
           CR                       := #CR,
           AUTO_OPEN                := L     21.2,
           AUTO_CLOSE               := L     21.3,
           FUSE                     := L     21.4,
           LS_OPEN                  := L     21.5,
           LS_CLOSE                 := L     21.6,
           ERROR_CONFIRM            := L     21.7,
           MAX_RUNTIME              := 180,
           OPEN                     := "R19-71VA21+19H3-K1.3:A1",
           CLOSE                    := "R19-71VA21+19H3-K1.2:A1",
           DDB                      := "DB_GRP_71".VA21);
      NOP   0;
NETWORK
TITLE ==71VA21-M1 CONTROL VALVE COOLING MODULE POSITION
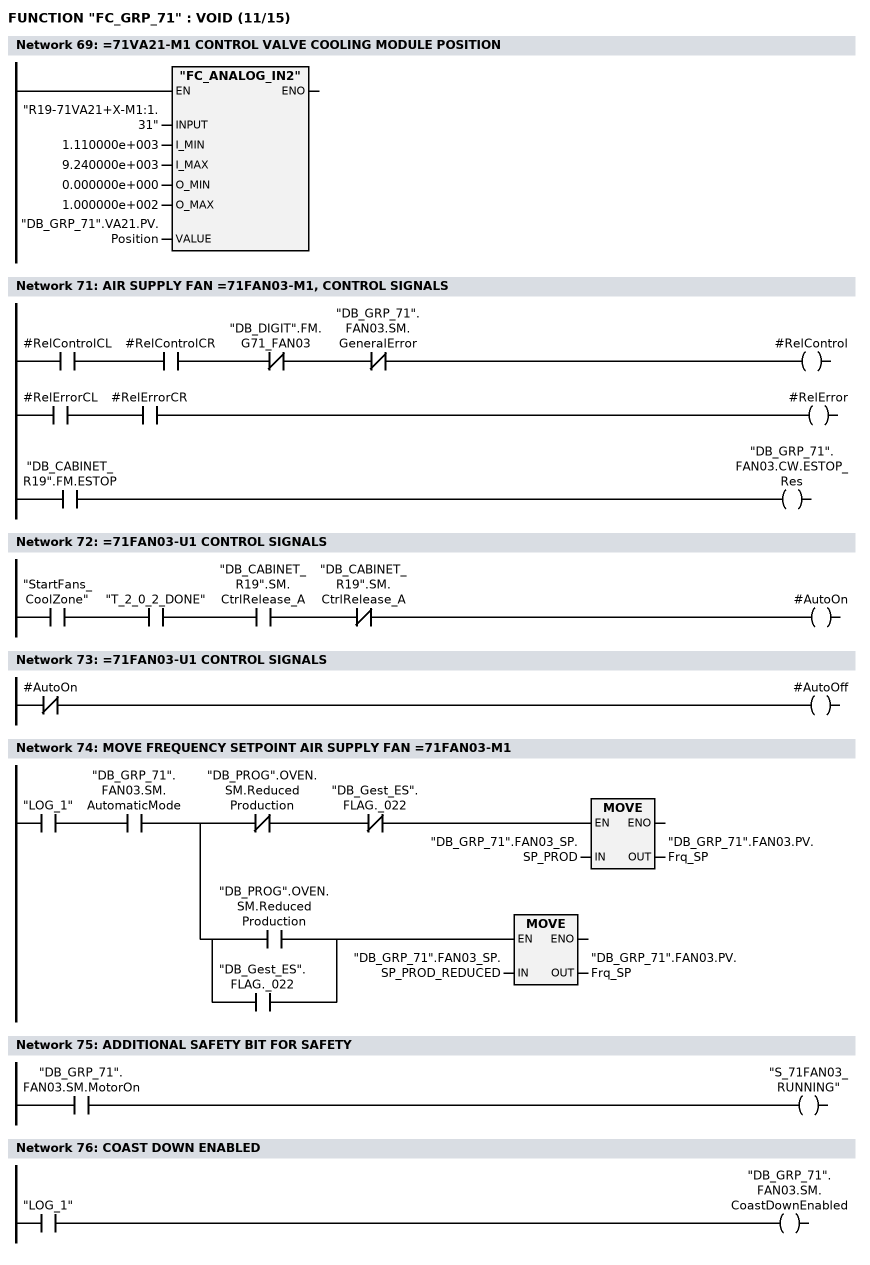
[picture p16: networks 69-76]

      CALL "FC_ANALOG_IN2" (
           INPUT                    := "R19-71VA21+X-M1:1.31",
           I_MIN                    := 1.110000e+003,
           I_MAX                    := 9.240000e+003,
           O_MIN                    := 0.000000e+000,
           O_MAX                    := 1.000000e+002,
           VALUE                    := "DB_GRP_71".VA21.PV.Position);
      NOP   0;
NETWORK
TITLE =*************** 31FAN03 **************

NETWORK
TITLE =AIR SUPPLY FAN =71FAN03-M1, CONTROL SIGNALS

      U     #RelControlCL;
      U     #RelControlCR;
      UN    "DB_DIGIT".FM.G71_FAN03;
      UN    "DB_GRP_71".FAN03.SM.GeneralError;
      =     #RelControl;

      U     #RelErrorCL;
      U     #RelErrorCR;
      =     #RelError;

      U     "DB_CABINET_R19".FM.ESTOP;
      =     "DB_GRP_71".FAN03.CW.ESTOP_Res;


NETWORK
TITLE ==71FAN03-U1 CONTROL SIGNALS

      U     "StartFans_CoolZone";
      U     "T_2_0_2_DONE";
      U     "DB_CABINET_R19".SM.CtrlRelease_A;
      UN    "DB_CABINET_R19".SM.CtrlRelease_A;
      =     #AutoOn;
NETWORK
TITLE ==71FAN03-U1 CONTROL SIGNALS

      UN    #AutoOn;
      =     #AutoOff;
NETWORK
TITLE =MOVE FREQUENCY SETPOINT AIR SUPPLY FAN =71FAN03-M1

      U     "LOG_1";
      U     "DB_GRP_71".FAN03.SM.AutomaticMode;
      =     L     21.0;
      U     L     21.0;
      UN    "DB_PROG".OVEN.SM.ReducedProduction;
      UN    "DB_Gest_ES".FLAG._022;
      SPBNB _003;
      L     "DB_GRP_71".FAN03_SP.SP_PROD;
      T     "DB_GRP_71".FAN03.PV.Frq_SP;
_003: NOP   0;
      U     L     21.0;
      U(    ;
      O     "DB_PROG".OVEN.SM.ReducedProduction;
      O     "DB_Gest_ES".FLAG._022;
      )     ;
      SPBNB _004;
      L     "DB_GRP_71".FAN03_SP.SP_PROD_REDUCED;
      T     "DB_GRP_71".FAN03.PV.Frq_SP;
_004: NOP   0;
NETWORK
TITLE =ADDITIONAL SAFETY BIT FOR SAFETY

      U     "DB_GRP_71".FAN03.SM.MotorOn;
      =     "S_71FAN03_RUNNING";
NETWORK
TITLE =COAST DOWN ENABLED

      U     "LOG_1";
      =     "DB_GRP_71".FAN03.SM.CoastDownEnabled;
NETWORK
TITLE ==71FAN03-U1 EXHAUST AIR FAN
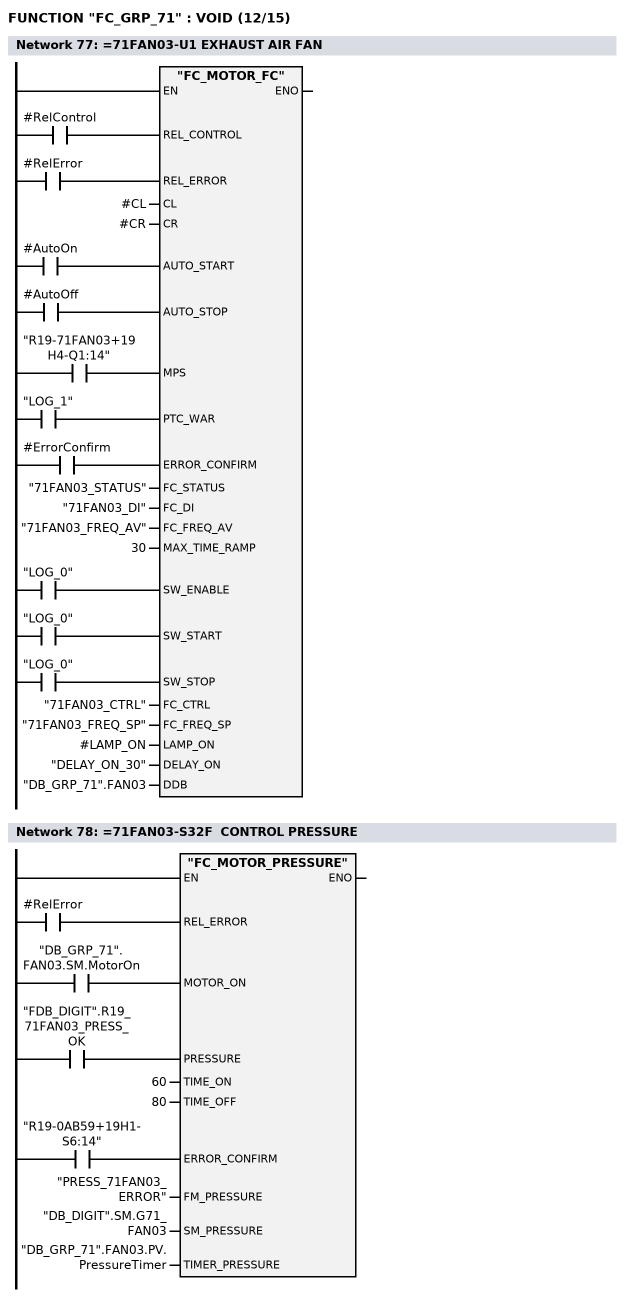
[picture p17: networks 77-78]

      U     #RelControl;
      =     L     21.0;
      BLD   103;
      U     #RelError;
      =     L     21.1;
      BLD   103;
      U     #AutoOn;
      =     L     21.2;
      BLD   103;
      U     #AutoOff;
      =     L     21.3;
      BLD   103;
      U     "R19-71FAN03+19H4-Q1:14";
      =     L     21.4;
      BLD   103;
      U     "LOG_1";
      =     L     21.5;
      BLD   103;
      U     #ErrorConfirm;
      =     L     21.6;
      BLD   103;
      U     "LOG_0";
      =     L     21.7;
      BLD   103;
      U     "LOG_0";
      =     L     22.0;
      BLD   103;
      U     "LOG_0";
      =     L     22.1;
      BLD   103;
      CALL "FC_MOTOR_FC" (
           REL_CONTROL              := L     21.0,
           REL_ERROR                := L     21.1,
           CL                       := #CL,
           CR                       := #CR,
           AUTO_START               := L     21.2,
           AUTO_STOP                := L     21.3,
           MPS                      := L     21.4,
           PTC_WAR                  := L     21.5,
           ERROR_CONFIRM            := L     21.6,
           FC_STATUS                := "71FAN03_STATUS",
           FC_DI                    := "71FAN03_DI",
           FC_FREQ_AV               := "71FAN03_FREQ_AV",
           MAX_TIME_RAMP            := 30,
           SW_ENABLE                := L     21.7,
           SW_START                 := L     22.0,
           SW_STOP                  := L     22.1,
           FC_CTRL                  := "71FAN03_CTRL",
           FC_FREQ_SP               := "71FAN03_FREQ_SP",
           LAMP_ON                  := #LAMP_ON,
           DELAY_ON                 := "DELAY_ON_30",
           DDB                      := "DB_GRP_71".FAN03);
      NOP   0;
NETWORK
TITLE ==71FAN03-S32F  CONTROL PRESSURE

      U     #RelError;
      =     L     21.0;
      BLD   103;
      U     "DB_GRP_71".FAN03.SM.MotorOn;
      =     L     21.1;
      BLD   103;
      U     "FDB_DIGIT".R19_71FAN03_PRESS_OK;
      =     L     21.2;
      BLD   103;
      U     "R19-0AB59+19H1-S6:14";
      =     L     21.3;
      BLD   103;
      CALL "FC_MOTOR_PRESSURE" (
           REL_ERROR                := L     21.0,
           MOTOR_ON                 := L     21.1,
           PRESSURE                 := L     21.2,
           TIME_ON                  := 60,
           TIME_OFF                 := 80,
           ERROR_CONFIRM            := L     21.3,
           FM_PRESSURE              := "PRESS_71FAN03_ERROR",
           SM_PRESSURE              := "DB_DIGIT".SM.G71_FAN03,
           TIMER_PRESSURE           := "DB_GRP_71".FAN03.PV.PressureTimer);
      NOP   0;
NETWORK
TITLE =PRESSURE ERROR =71FAN03
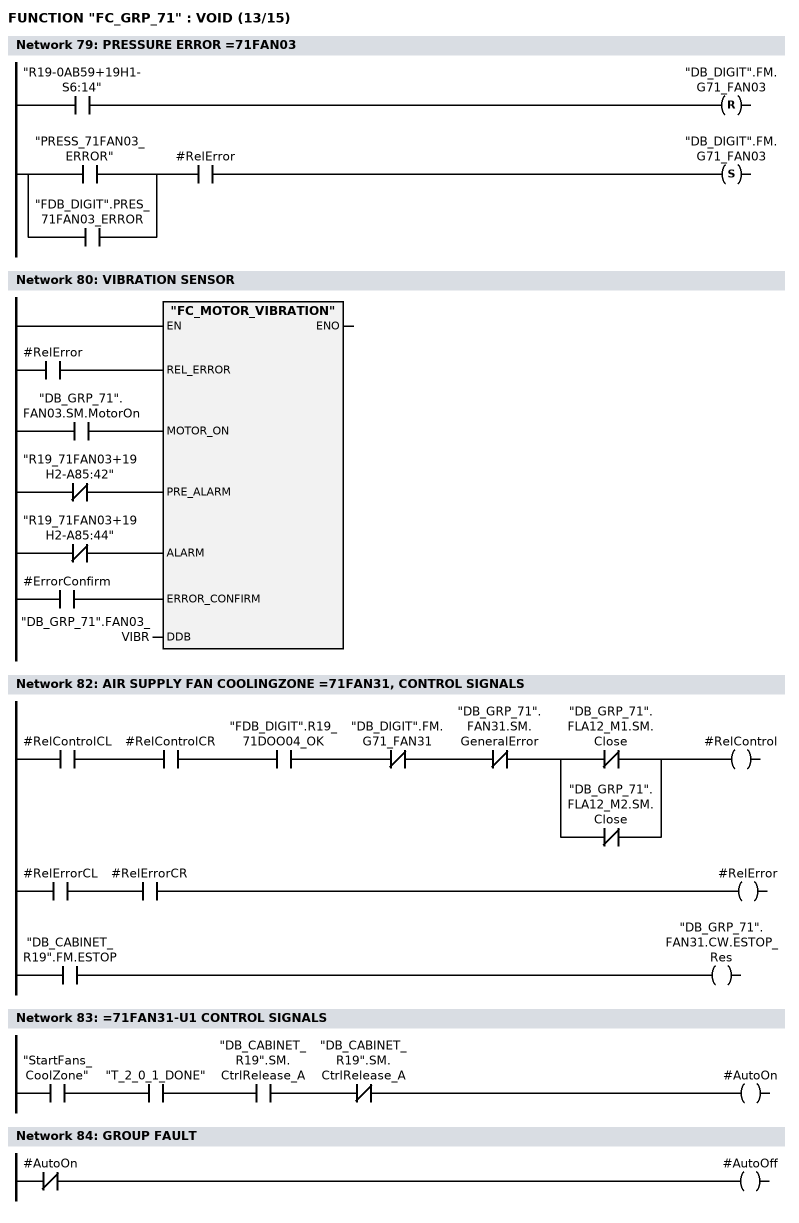
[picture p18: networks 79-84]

      U     "R19-0AB59+19H1-S6:14";
      R     "DB_DIGIT".FM.G71_FAN03;
      U(    ;
      O     "PRESS_71FAN03_ERROR";
      O     "FDB_DIGIT".PRES_71FAN03_ERROR;
      )     ;
      U     #RelError;
      S     "DB_DIGIT".FM.G71_FAN03;
      NOP   0;
NETWORK
TITLE =VIBRATION SENSOR

      U     #RelError;
      =     L     21.0;
      BLD   103;
      U     "DB_GRP_71".FAN03.SM.MotorOn;
      =     L     21.1;
      BLD   103;
      UN    "R19_71FAN03+19H2-A85:42";
      =     L     21.2;
      BLD   103;
      UN    "R19_71FAN03+19H2-A85:44";
      =     L     21.3;
      BLD   103;
      U     #ErrorConfirm;
      =     L     21.4;
      BLD   103;
      CALL "FC_MOTOR_VIBRATION" (
           REL_ERROR                := L     21.0,
           MOTOR_ON                 := L     21.1,
           PRE_ALARM                := L     21.2,
           ALARM                    := L     21.3,
           ERROR_CONFIRM            := L     21.4,
           DDB                      := "DB_GRP_71".FAN03_VIBR);
      NOP   0;
NETWORK
TITLE =************** 71FAN31 ****************

NETWORK
TITLE =AIR SUPPLY FAN COOLINGZONE =71FAN31, CONTROL SIGNALS

      U     #RelControlCL;
      U     #RelControlCR;
      U     "FDB_DIGIT".R19_71DOO04_OK;
      UN    "DB_DIGIT".FM.G71_FAN31;
      UN    "DB_GRP_71".FAN31.SM.GeneralError;
      U(    ;
      ON    "DB_GRP_71".FLA12_M1.SM.Close;
      ON    "DB_GRP_71".FLA12_M2.SM.Close;
      )     ;
      =     #RelControl;


      U     #RelErrorCL;
      U     #RelErrorCR;
      =     #RelError;

      U     "DB_CABINET_R19".FM.ESTOP;
      =     "DB_GRP_71".FAN31.CW.ESTOP_Res;


NETWORK
TITLE ==71FAN31-U1 CONTROL SIGNALS

      U     "StartFans_CoolZone";
      U     "T_2_0_1_DONE";
      U     "DB_CABINET_R19".SM.CtrlRelease_A;
      UN    "DB_CABINET_R19".SM.CtrlRelease_A;
      =     #AutoOn;
NETWORK
TITLE =GROUP FAULT

      UN    #AutoOn;
      =     #AutoOff;
NETWORK
TITLE =MOVE FREQUENCY SETPOINT TO AIR SUPPLY FAN COOLINGZONE =71FAN31
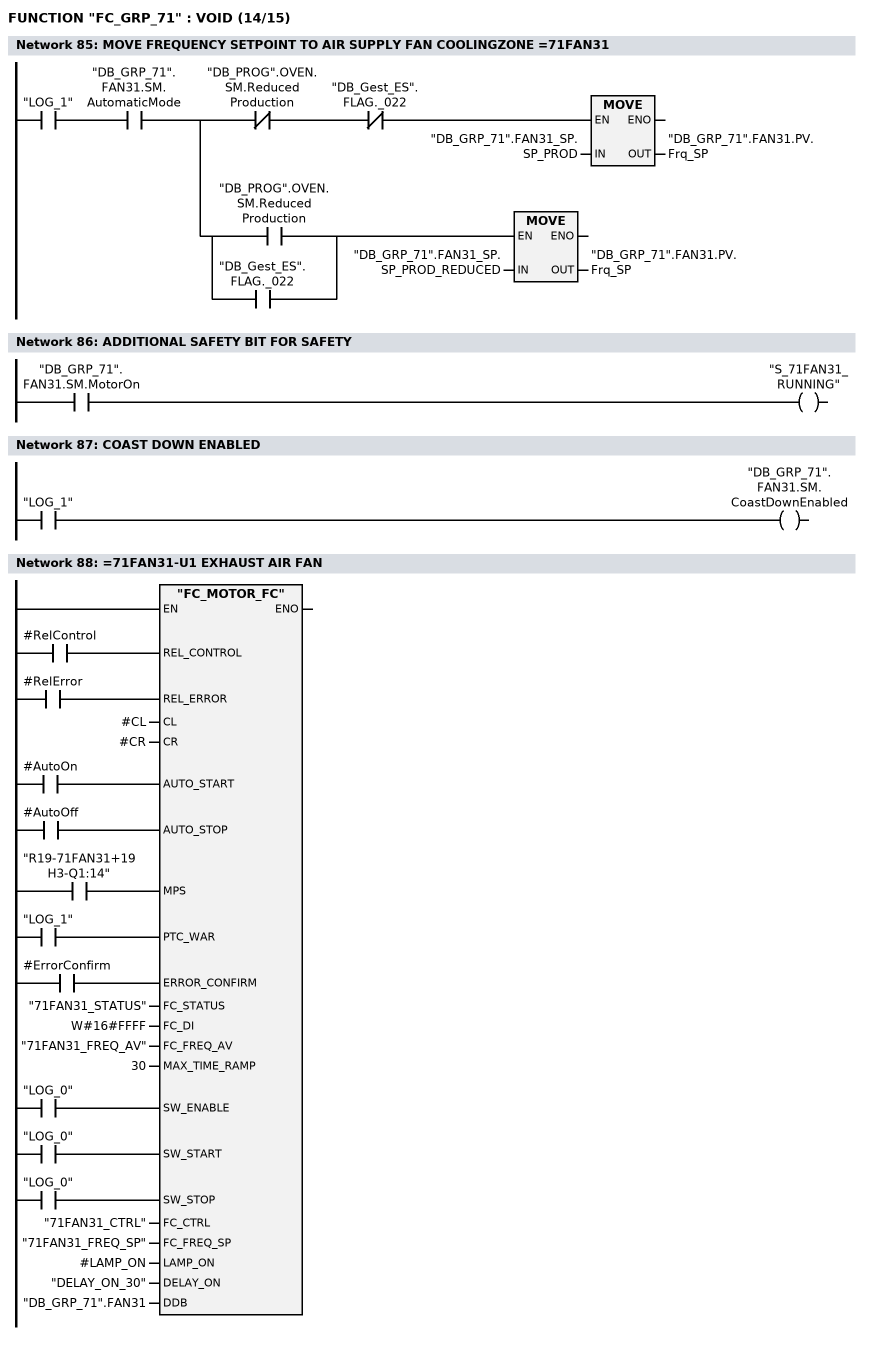
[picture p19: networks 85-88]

      U     "LOG_1";
      U     "DB_GRP_71".FAN31.SM.AutomaticMode;
      =     L     21.0;
      U     L     21.0;
      UN    "DB_PROG".OVEN.SM.ReducedProduction;
      UN    "DB_Gest_ES".FLAG._022;
      SPBNB _005;
      L     "DB_GRP_71".FAN31_SP.SP_PROD;
      T     "DB_GRP_71".FAN31.PV.Frq_SP;
_005: NOP   0;
      U     L     21.0;
      U(    ;
      O     "DB_PROG".OVEN.SM.ReducedProduction;
      O     "DB_Gest_ES".FLAG._022;
      )     ;
      SPBNB _006;
      L     "DB_GRP_71".FAN31_SP.SP_PROD_REDUCED;
      T     "DB_GRP_71".FAN31.PV.Frq_SP;
_006: NOP   0;
NETWORK
TITLE =ADDITIONAL SAFETY BIT FOR SAFETY

      U     "DB_GRP_71".FAN31.SM.MotorOn;
      =     "S_71FAN31_RUNNING";
NETWORK
TITLE =COAST DOWN ENABLED

      U     "LOG_1";
      =     "DB_GRP_71".FAN31.SM.CoastDownEnabled;
NETWORK
TITLE ==71FAN31-U1 EXHAUST AIR FAN

      U     #RelControl;
      =     L     21.0;
      BLD   103;
      U     #RelError;
      =     L     21.1;
      BLD   103;
      U     #AutoOn;
      =     L     21.2;
      BLD   103;
      U     #AutoOff;
      =     L     21.3;
      BLD   103;
      U     "R19-71FAN31+19H3-Q1:14";
      =     L     21.4;
      BLD   103;
      U     "LOG_1";
      =     L     21.5;
      BLD   103;
      U     #ErrorConfirm;
      =     L     21.6;
      BLD   103;
      U     "LOG_0";
      =     L     21.7;
      BLD   103;
      U     "LOG_0";
      =     L     22.0;
      BLD   103;
      U     "LOG_0";
      =     L     22.1;
      BLD   103;
      CALL "FC_MOTOR_FC" (
           REL_CONTROL              := L     21.0,
           REL_ERROR                := L     21.1,
           CL                       := #CL,
           CR                       := #CR,
           AUTO_START               := L     21.2,
           AUTO_STOP                := L     21.3,
           MPS                      := L     21.4,
           PTC_WAR                  := L     21.5,
           ERROR_CONFIRM            := L     21.6,
           FC_STATUS                := "71FAN31_STATUS",
           FC_DI                    := W#16#FFFF,
           FC_FREQ_AV               := "71FAN31_FREQ_AV",
           MAX_TIME_RAMP            := 30,
           SW_ENABLE                := L     21.7,
           SW_START                 := L     22.0,
           SW_STOP                  := L     22.1,
           FC_CTRL                  := "71FAN31_CTRL",
           FC_FREQ_SP               := "71FAN31_FREQ_SP",
           LAMP_ON                  := #LAMP_ON,
           DELAY_ON                 := "DELAY_ON_30",
           DDB                      := "DB_GRP_71".FAN31);
      NOP   0;
NETWORK
TITLE ==71FAN31-S32F  CONTROL PRESSURE
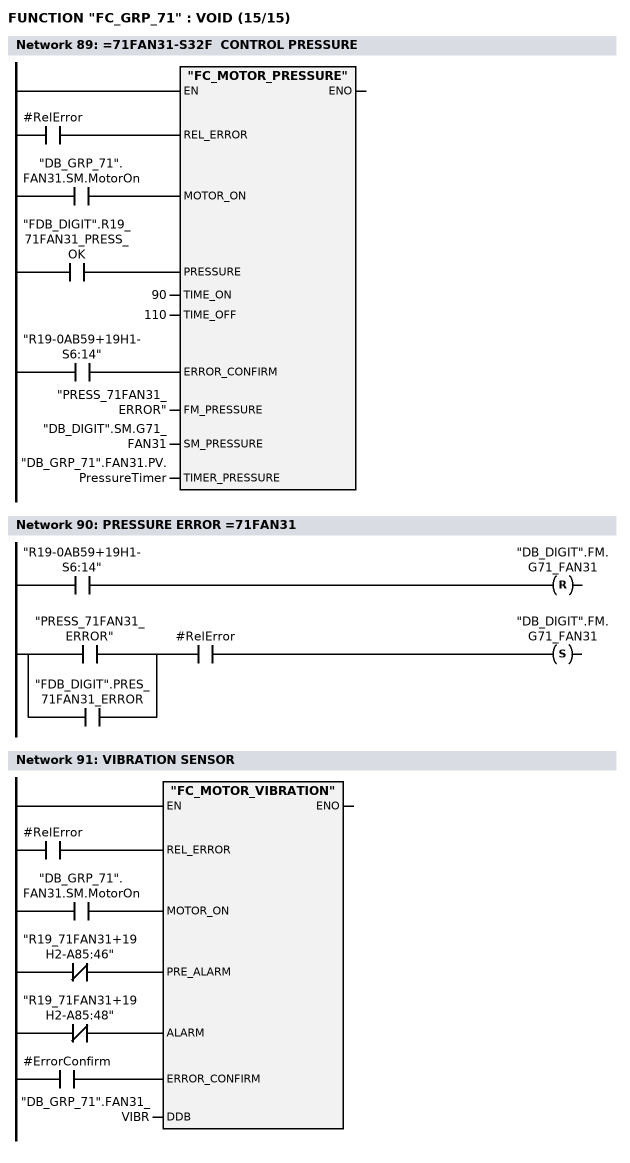
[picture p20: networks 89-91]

      U     #RelError;
      =     L     21.0;
      BLD   103;
      U     "DB_GRP_71".FAN31.SM.MotorOn;
      =     L     21.1;
      BLD   103;
      U     "FDB_DIGIT".R19_71FAN31_PRESS_OK;
      =     L     21.2;
      BLD   103;
      U     "R19-0AB59+19H1-S6:14";
      =     L     21.3;
      BLD   103;
      CALL "FC_MOTOR_PRESSURE" (
           REL_ERROR                := L     21.0,
           MOTOR_ON                 := L     21.1,
           PRESSURE                 := L     21.2,
           TIME_ON                  := 90,
           TIME_OFF                 := 110,
           ERROR_CONFIRM            := L     21.3,
           FM_PRESSURE              := "PRESS_71FAN31_ERROR",
           SM_PRESSURE              := "DB_DIGIT".SM.G71_FAN31,
           TIMER_PRESSURE           := "DB_GRP_71".FAN31.PV.PressureTimer);
      NOP   0;
NETWORK
TITLE =PRESSURE ERROR =71FAN31

      U     "R19-0AB59+19H1-S6:14";
      R     "DB_DIGIT".FM.G71_FAN31;
      U(    ;
      O     "PRESS_71FAN31_ERROR";
      O     "FDB_DIGIT".PRES_71FAN31_ERROR;
      )     ;
      U     #RelError;
      S     "DB_DIGIT".FM.G71_FAN31;
      NOP   0;
NETWORK
TITLE =VIBRATION SENSOR

      U     #RelError;
      =     L     21.0;
      BLD   103;
      U     "DB_GRP_71".FAN31.SM.MotorOn;
      =     L     21.1;
      BLD   103;
      UN    "R19_71FAN31+19H2-A85:46";
      =     L     21.2;
      BLD   103;
      UN    "R19_71FAN31+19H2-A85:48";
      =     L     21.3;
      BLD   103;
      U     #ErrorConfirm;
      =     L     21.4;
      BLD   103;
      CALL "FC_MOTOR_VIBRATION" (
           REL_ERROR                := L     21.0,
           MOTOR_ON                 := L     21.1,
           PRE_ALARM                := L     21.2,
           ALARM                    := L     21.3,
           ERROR_CONFIRM            := L     21.4,
           DDB                      := "DB_GRP_71".FAN31_VIBR);
      NOP   0;
NETWORK
TITLE =END



END_FUNCTION

